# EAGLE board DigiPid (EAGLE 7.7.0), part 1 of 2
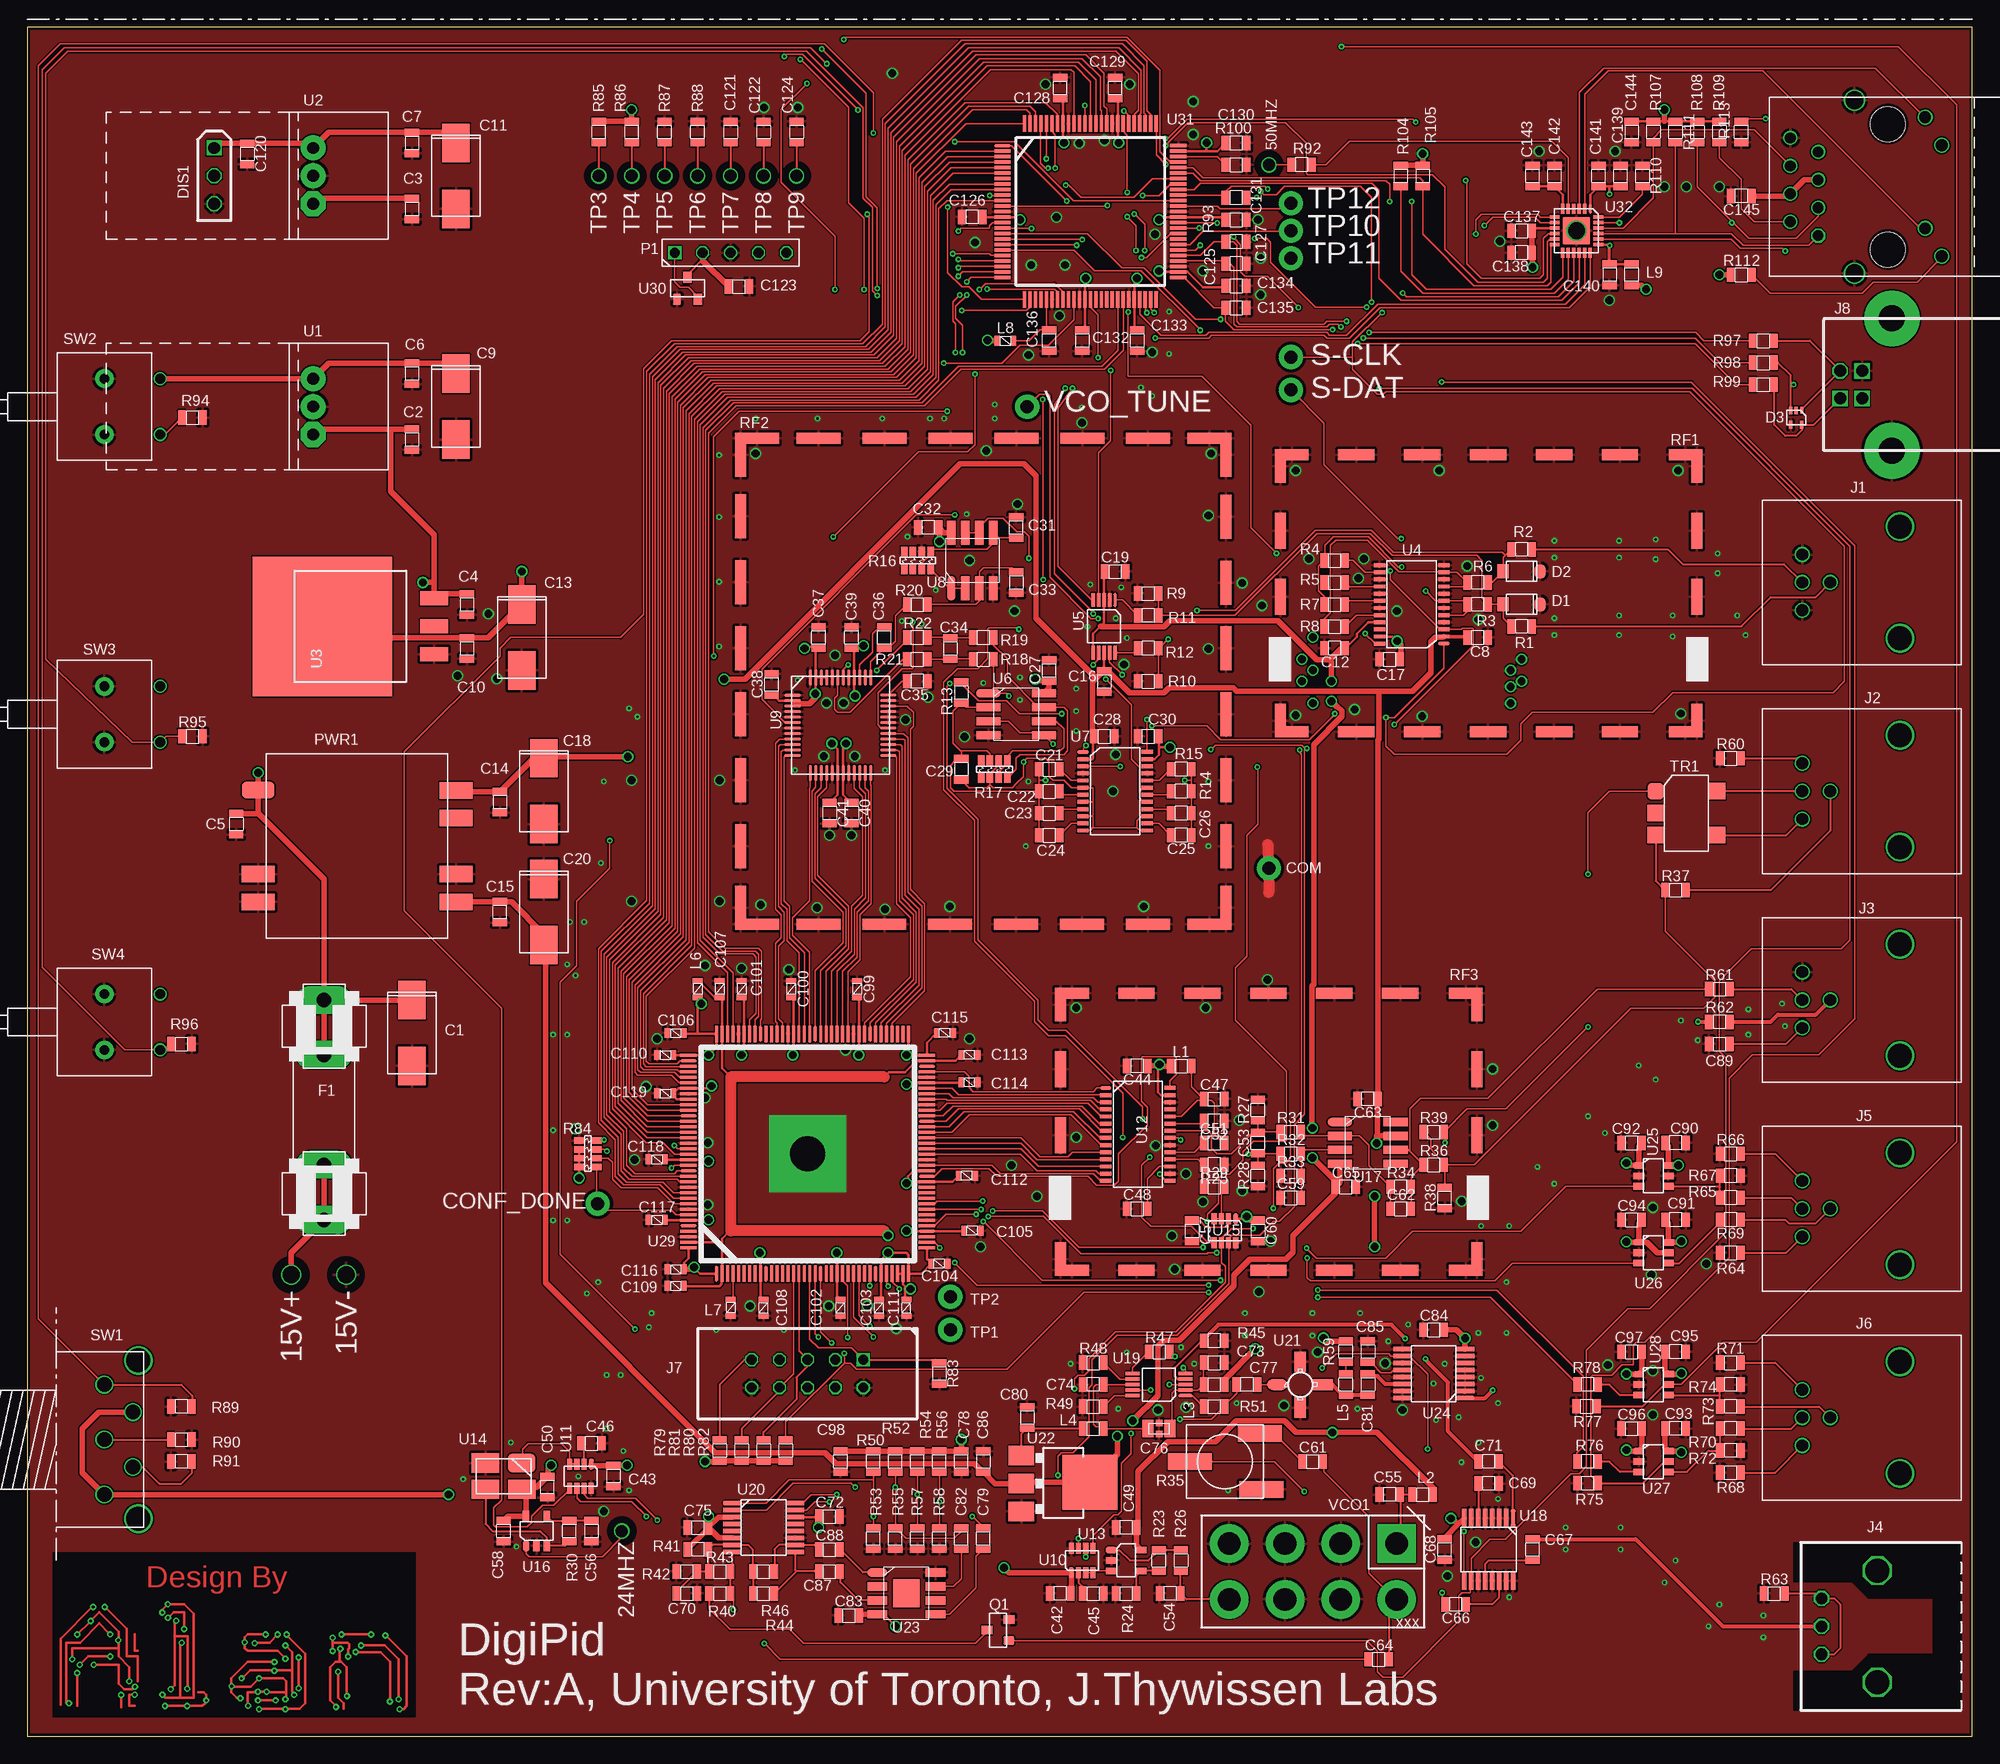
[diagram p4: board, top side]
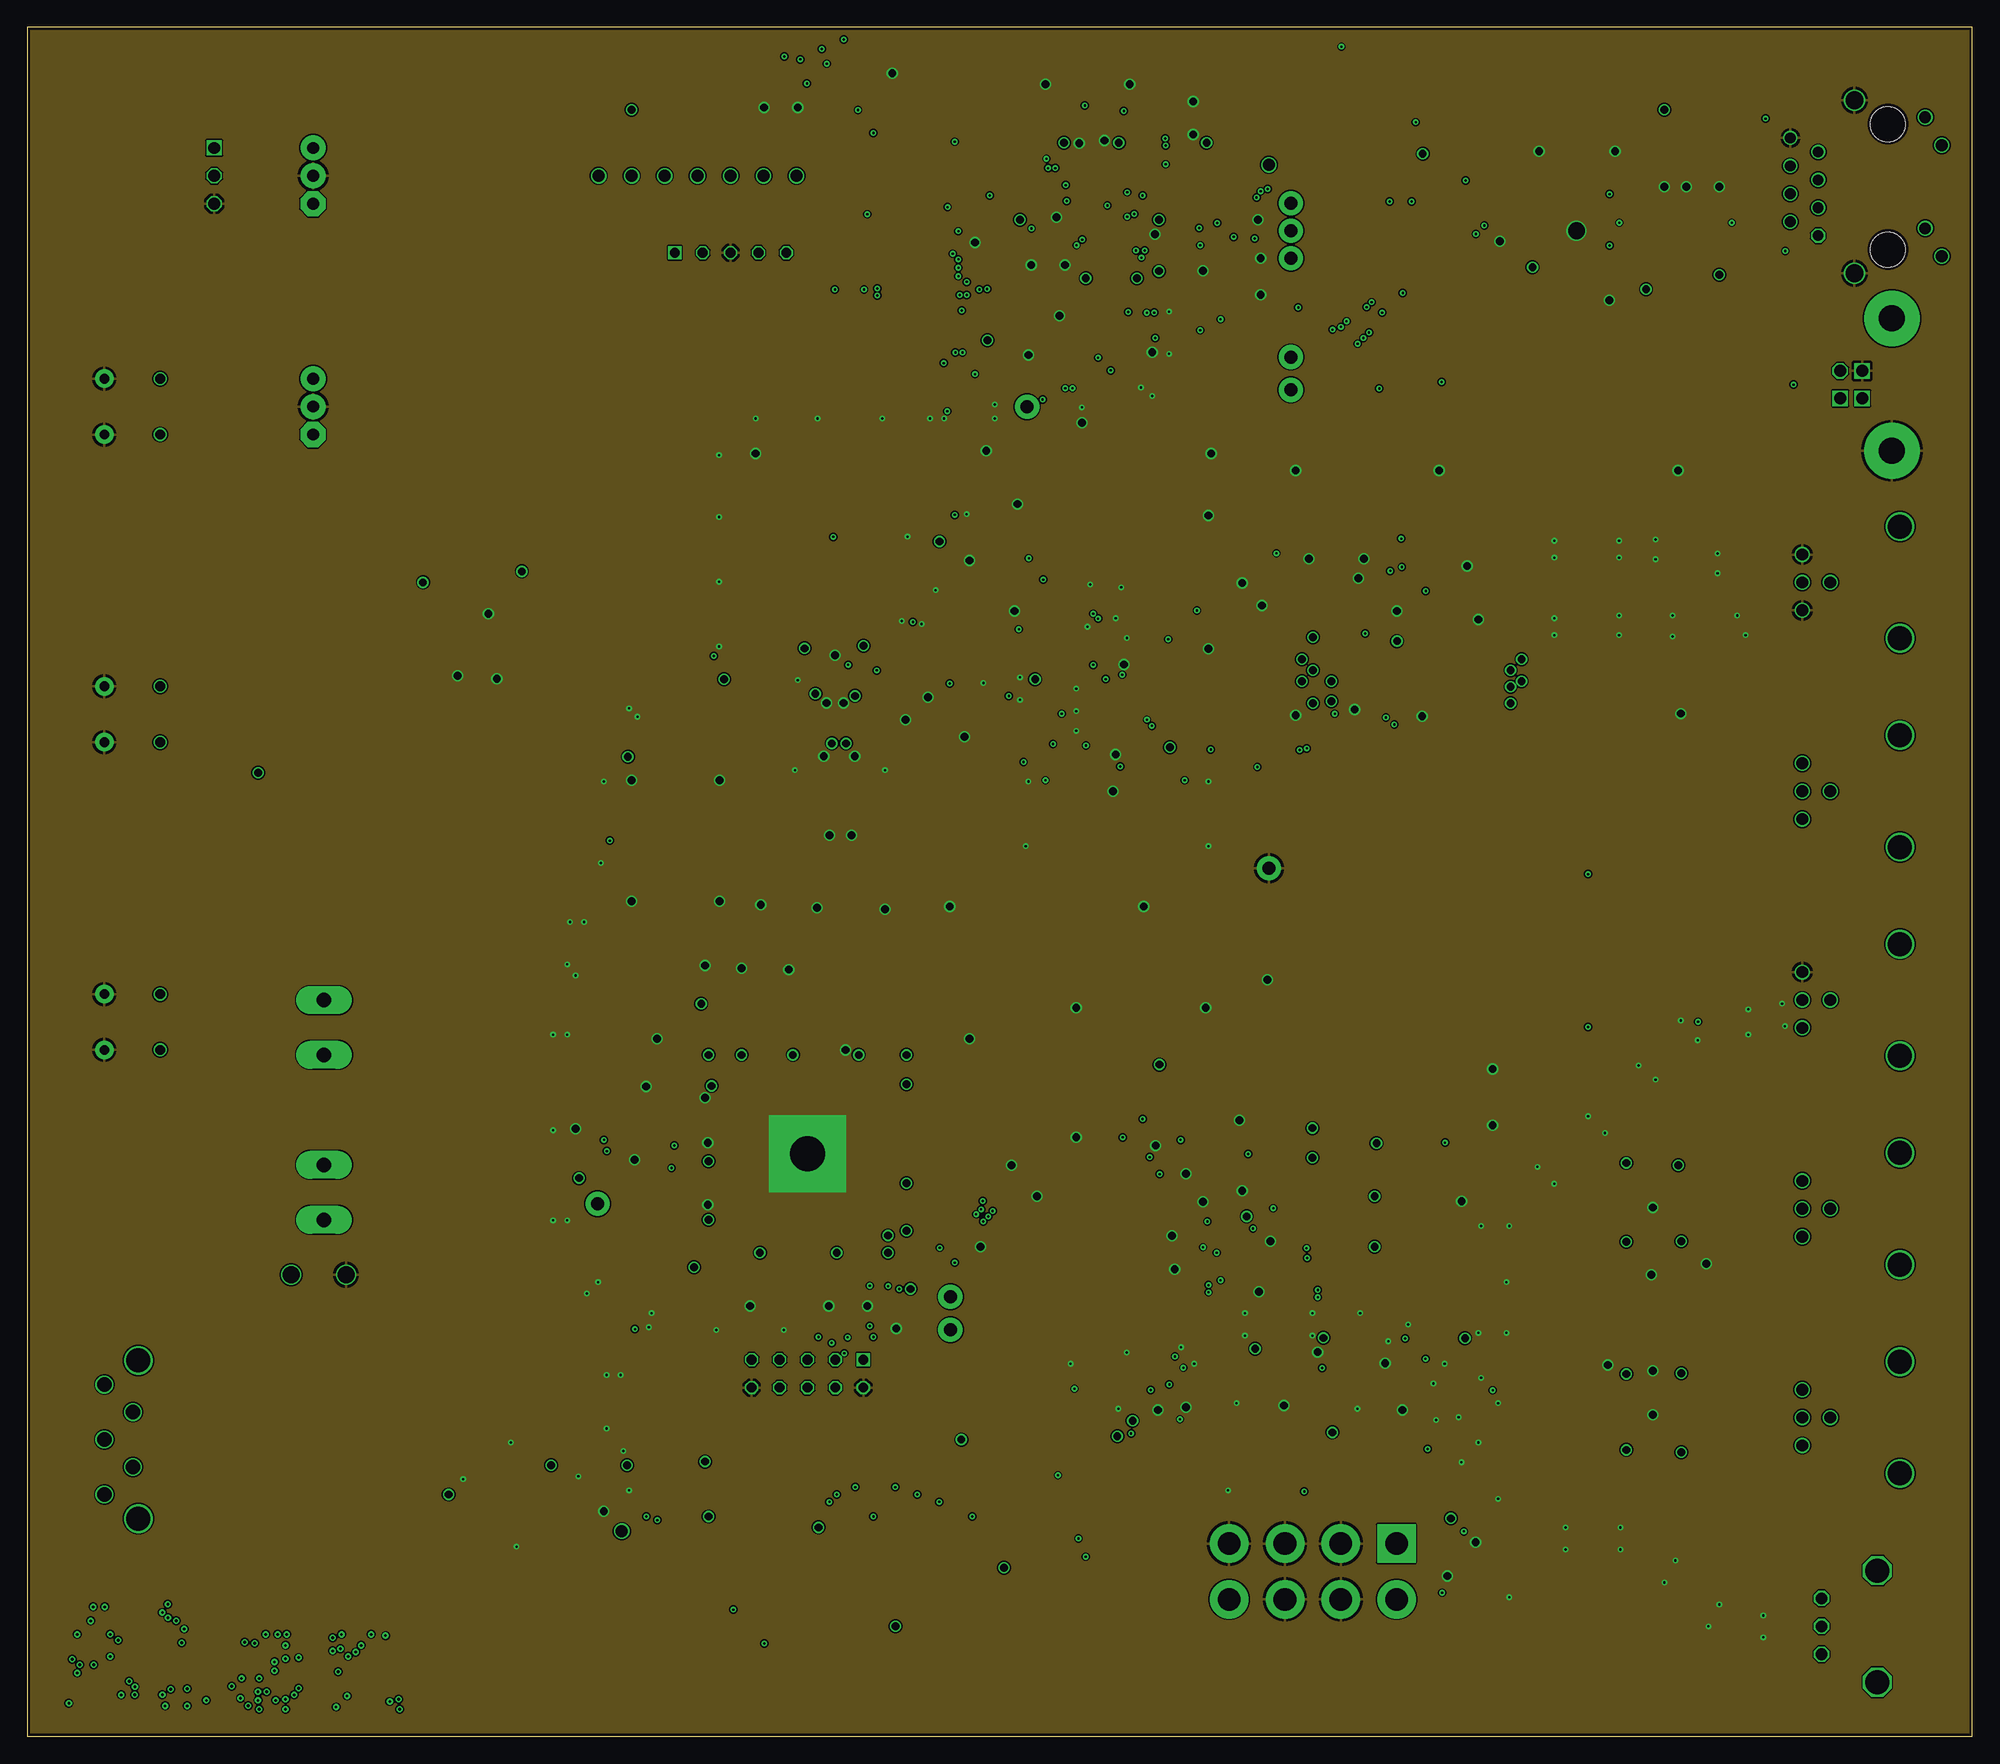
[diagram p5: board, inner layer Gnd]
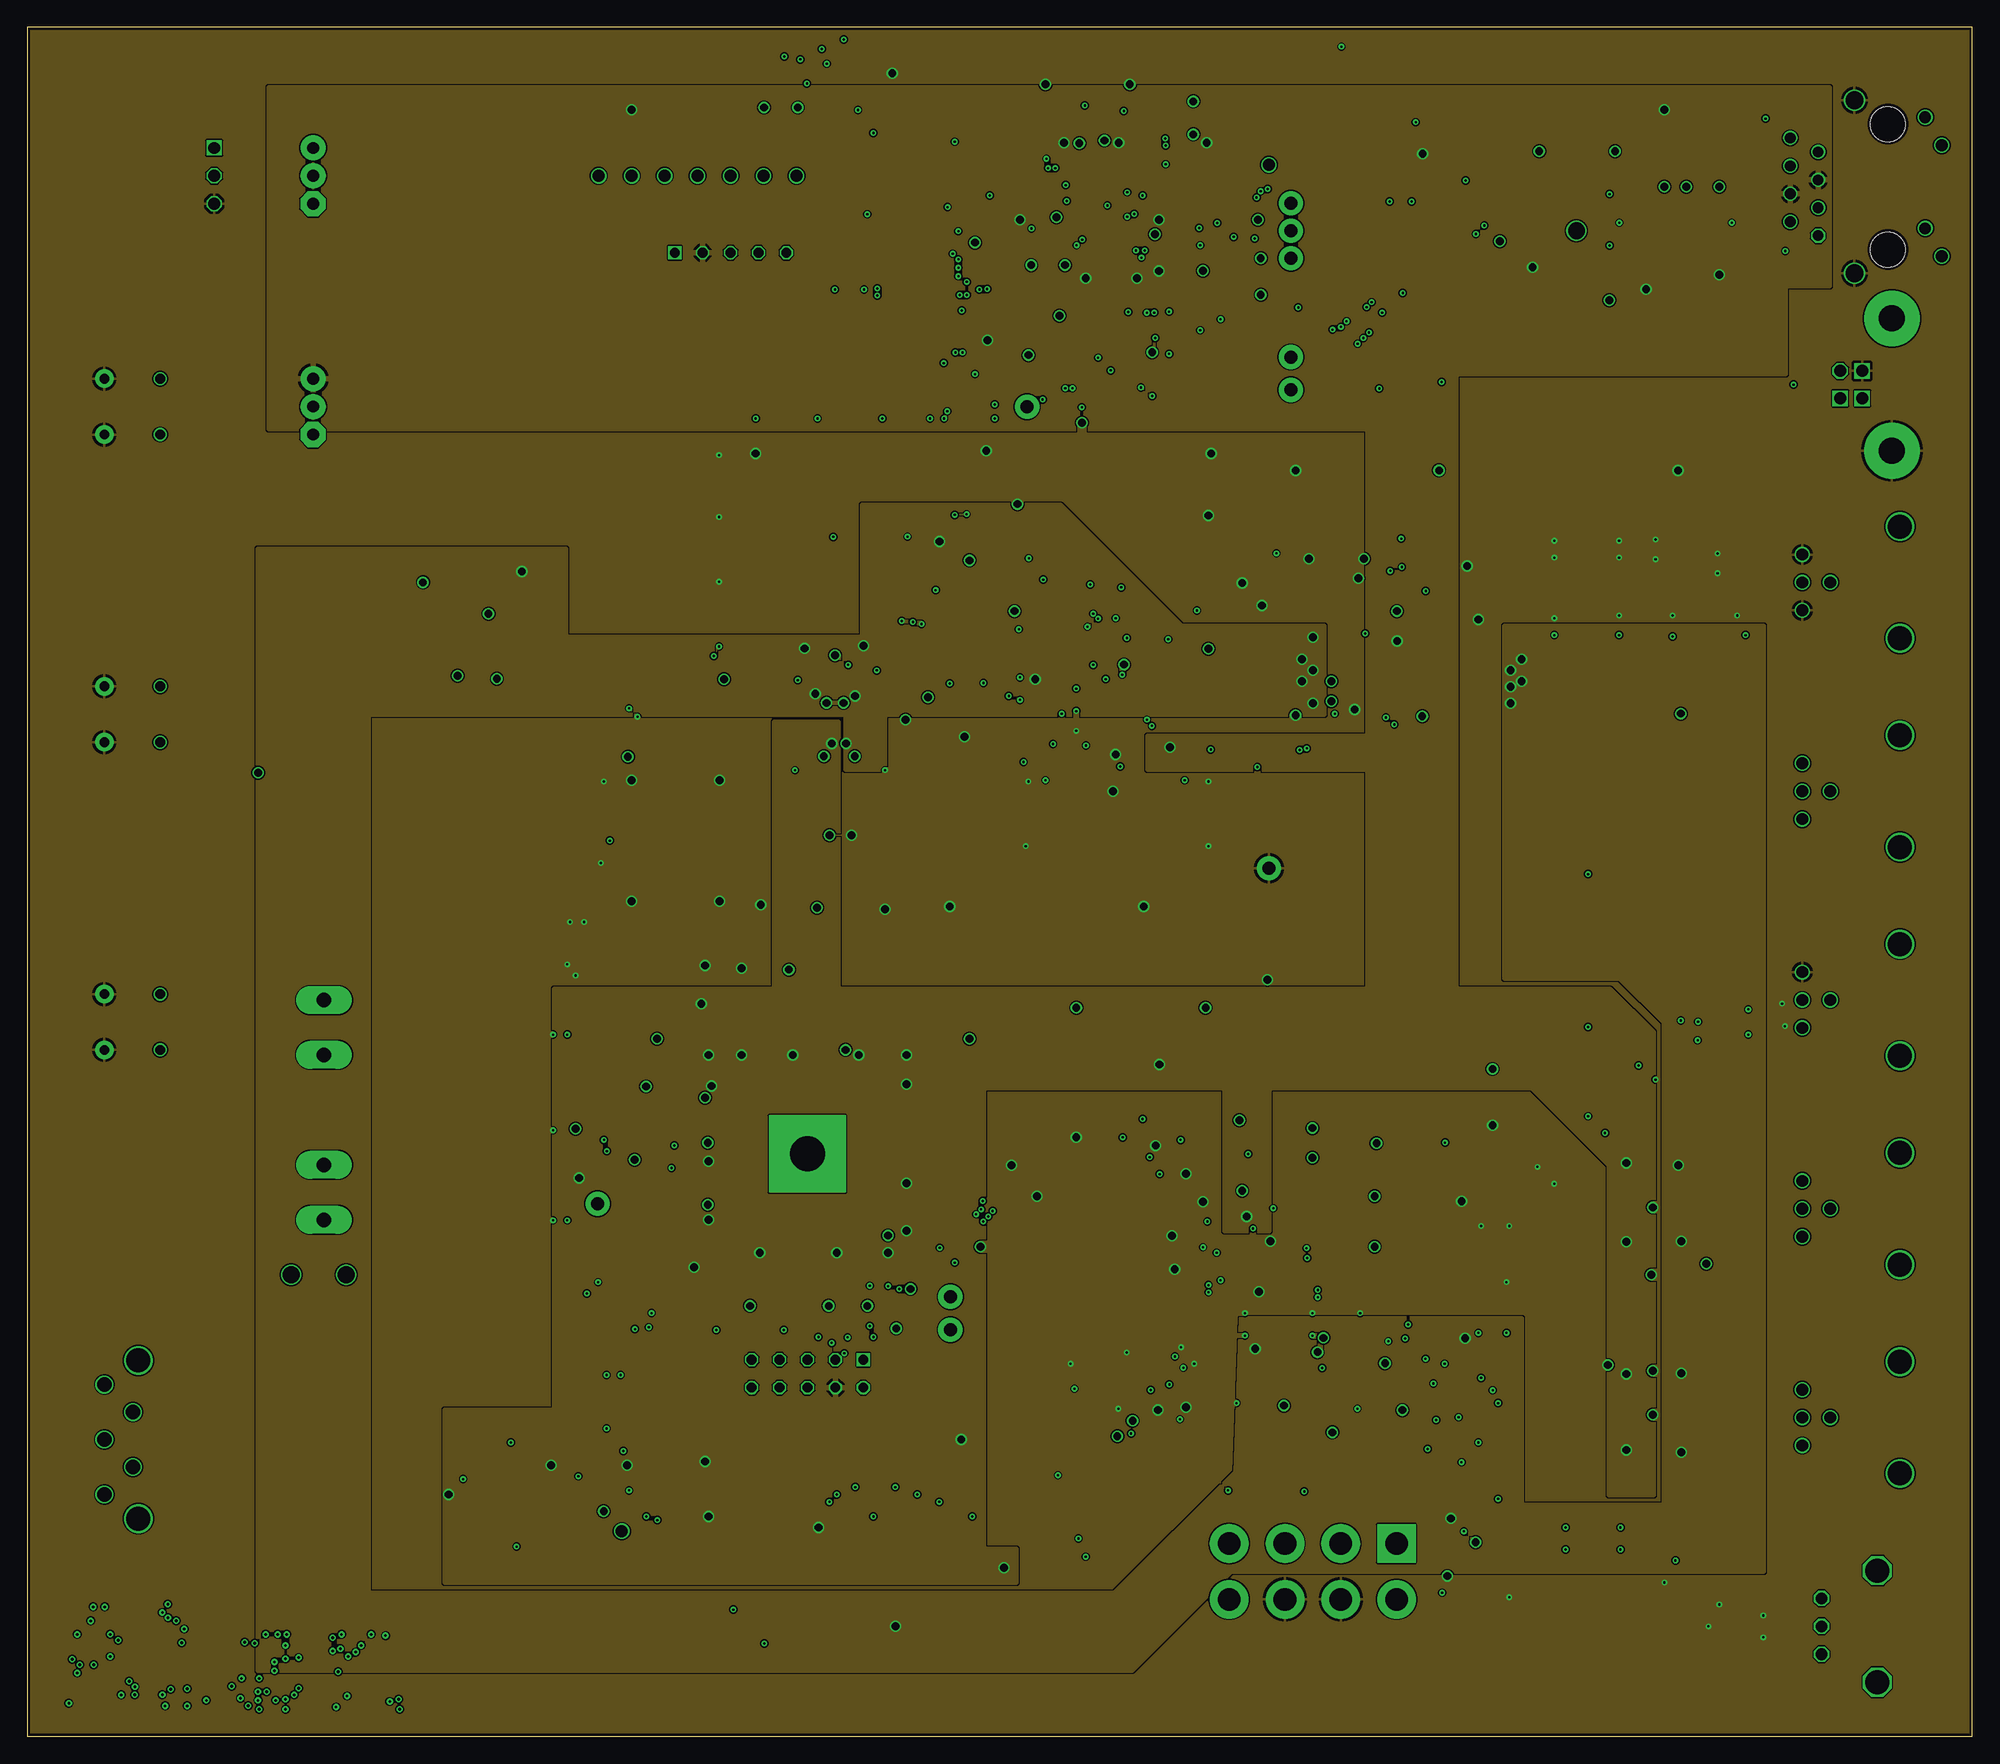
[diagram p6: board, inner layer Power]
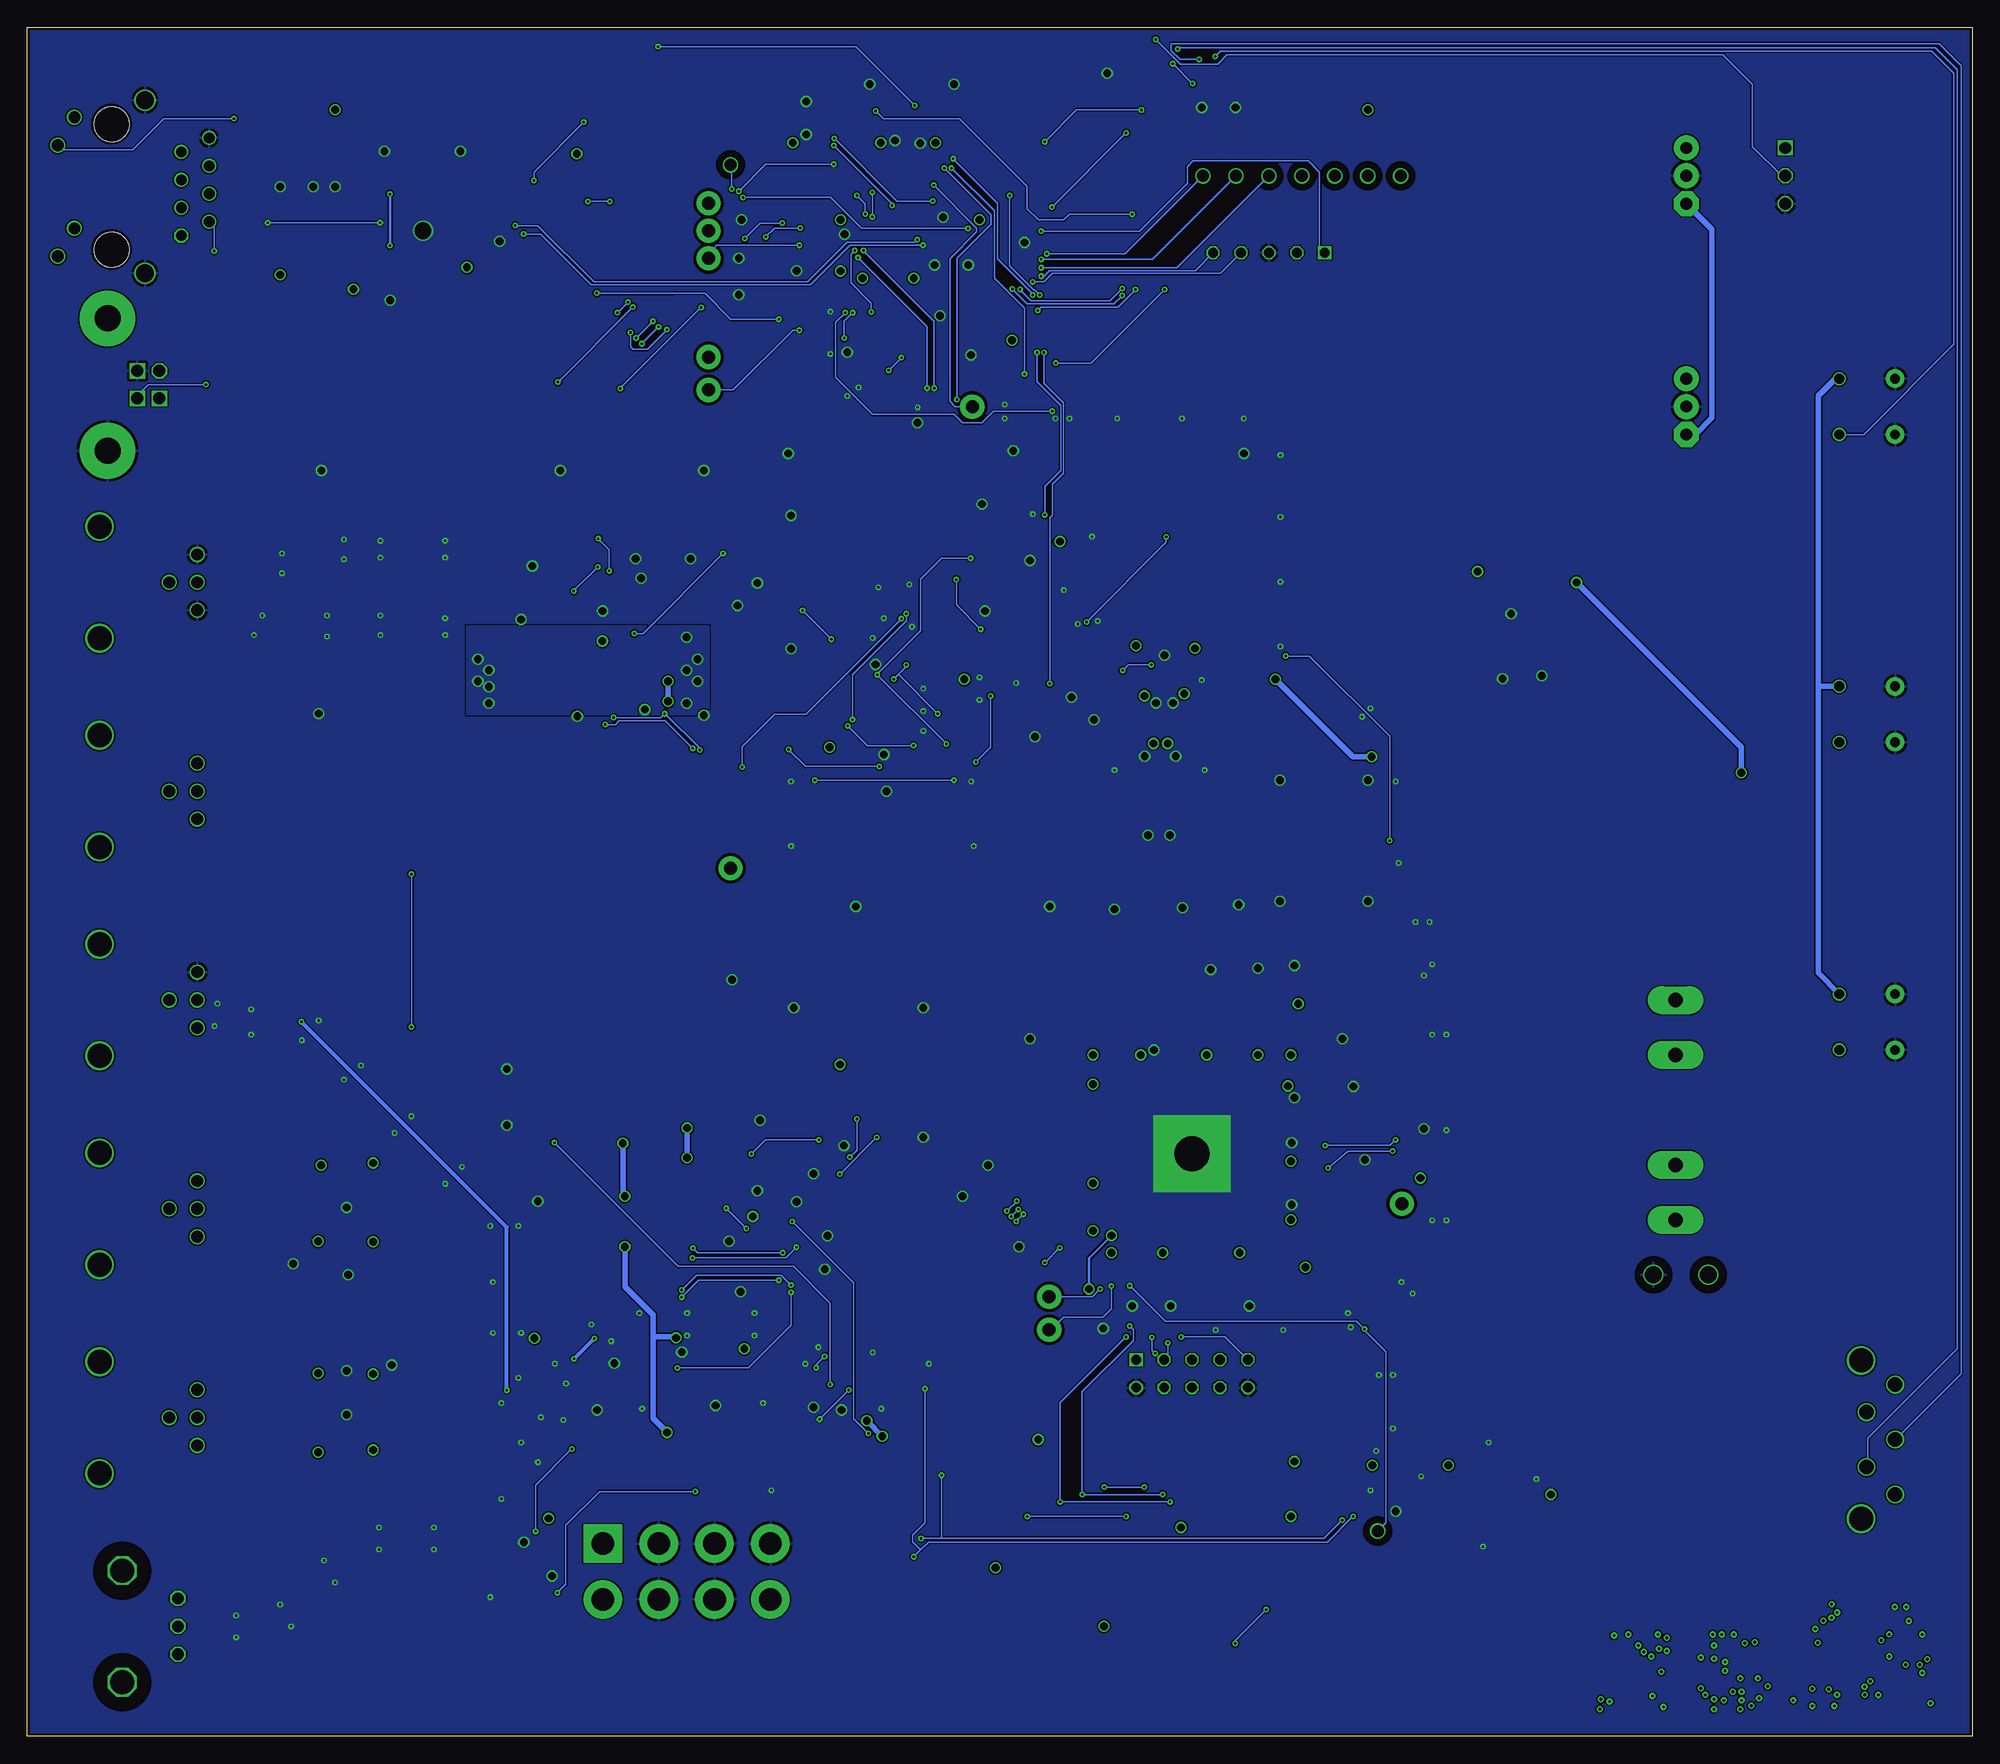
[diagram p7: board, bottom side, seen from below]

Size 177 x 155.5 mm. Coordinates in mm from the lower left corner, seen from the top.
Outline: 0,0 177,0 177,155.5 0,155.5 0,0
Copper layers (1+2+3+16): Top 0.04318125mm / dielectric 7.5mil / Gnd 0.035559375mm / dielectric 40mil / Power 0.035559375mm / dielectric 7.5mil / Bottom 0.04318125mm
Design rules "~DRC for Pentalogix, 4-layer": minimum track width 5mil, minimum drill 8mil, track to track 5mil, track to pad 5mil, pad to pad 5mil, via to via 5mil, smd to smd 0mil, copper to edge 10mil, drill to drill 5mil, minimum pad ring 6mil, minimum via ring 6mil, stop-mask expansion 4mil, vias tented up to drill 0mil, thermal gap 10mil
Net classes: 0 default: width 0.127 mm, drill 0.203 mm, clearance 0.127 mm; 1 Power: width 0.25 mm, drill 0.711 mm, clearance 0.127 mm; 2 Microstrip_50: width 0.356 mm, clearance 0.508 mm; 3 Power,0.25mm: width 0.25 mm, drill 0.711 mm, clearance 0.127 mm
tRestrict: 4 lines

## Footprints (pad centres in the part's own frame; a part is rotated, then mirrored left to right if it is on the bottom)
TP,1.5MM = drill 1.524: TP 0,0
TP-0.042B = drill 1.092: TP 0,0
7343 = smd 3.5 x 2.5: +VE -3,0; -VE 3,0
2012(0805) = smd 0.7 x 1.3: 1 -0.95,0; 2 0.95,0
1608(0603)X2Y_DUAL = smd 1 x 1.6: 1 -1,0; 2 1,0 | smd 0.6 x 0.6: COM1 0,-0.5; COM2 0,0.5
1608(0603) = smd 0.5 x 0.9: 1 -0.75,0; 2 0.75,0
TP-0.042C = drill 1.181 pad 2.2: TP 0,0
SOD123 = smd 1.016 x 1.27: A 1.676,0; C -1.676,0
SOT553 = smd 0.323 x 0.7: 1 -0.503,-0.65; 2 0,-0.65; 3 0.503,-0.65; 4 0.5,0.65; 5 -0.5,0.65
DISPLAY:3WIRE = drill 1.067 octagon: COM 0,-2.54; RXD 0,0 | drill 1.067 square: VDD 0,2.54
FUSE = drill 1.321 pad 2.54 long: 1A -10,0; 1B -5,0; 2A 10,0; 2B 5,0
CONN:BNC,DUAL(BOMAR) = drill 1.067: LWR-COM 14.45,-2.54; LWR-CTR 11.91,0; UPR-COM 14.45,2.54; UPR-CTR 14.45,0 | drill 2.184: MTG1 5.56,-5.08; MTG2 5.56,5.08
CONN:BNC-AMP-TYPE3HORIZ = drill 1.067 octagon: CONDUCTOR 0,-12.7; SHIELD1 -2.54,-12.7; SHIELD2 2.54,-12.7 | drill 2.184 octagon: P$1 -5.08,-7.62; P$2 5.08,-7.62
CONN:2X5-BLASTER = drill 0.889 square: 1 -1.27,5.08 | drill 0.889 octagon: 2 1.27,5.08; 3 -1.27,2.54; 4 1.27,2.54; 5 -1.27,0; 6 1.27,0; 7 -1.27,-2.54; 8 1.27,-2.54; 9 -1.27,-5.08; 10 1.27,-5.08
CONN,USB_AU-Y1007 = drill 1.092 octagon: 1 1.25,0 | drill 1.092 square: 2 -1.25,0; 3 -1.25,-2; 4 1.25,-2 | drill 2.362 pad 5.08: S1 -6.02,-4.71; S2 6.02,-4.71
CONN,1X5,100MIL = drill 0.889 square: 1 0,5.08 | drill 0.889 octagon: 2 0,2.54; 3 0,0; 4 0,-2.54; 5 0,-5.08
CONN,RJ45_WITH_MAGNETICS_LEDS#1 = drill 0.965 octagon: 1 4.445,0 | drill 0.965: 2 3.175,-2.54; 3 1.905,0; 4 0.635,-2.54; 5 -0.635,0; 6 -1.905,-2.54; 7 -3.175,0; 8 -4.445,-2.54 | drill 1.067: 9 6.325,11.252; 10 3.785,9.728; 11 -3.785,11.252; 12 -6.325,9.728 | drill 1.613: SHLD1 7.874,3.302; SHLD2 -7.874,3.302 | hole 3.175: 5.715,6.35; -5.715,6.35
DC-DC:CC1R5-XXXXX-R-E(TDK/LAMBDA) = smd 3 x 1.5: +VIN -9,5.1; +VOUT 9,5.08; -VIN -9,-5.08; -VOUT 9,-5.08; COM 9,-2.54; RC -9,-2.54; TRM 9,2.54
SOT23 = smd 0.75 x 1: 1 -0.95,-1; 2 0.95,-1; 3 0,1
PANASONIC_EXB-V8V(QUAD-R-PACK) = smd 0.9 x 0.59: 1A -0.8,1.2; 1B 0.8,1.2; 2A -0.8,0.4; 2B 0.8,0.4; 3A -0.8,-0.4; 3B 0.8,-0.4; 4A -0.8,-1.2; 4B 0.8,-1.2
BOURNS_3361P = smd 1.5 x 4: CCW -2.54,-3.3; CW 2.54,-3.2; W 0,3.2
RF-SHIELD,38X25MM(BMI-S-205-F) = smd 3.3 x 1: 1 -5.7,-18.95; 2 0.3,-18.95; 5 -5.7,18.95; 7 0.3,18.95 | smd 2.7 x 1: 3 6,-18.95; 8 6,18.95 | smd 3.05 x 1: 4 11.575,-18.95; 6 -11.575,18.95; 9 11.575,18.95; 25 -11.575,-18.95 | smd 1 x 3.3: 10 -12.6,-12.05; 12 -12.6,-6.05; 13 -12.6,-0.05; 15 12.6,-12.05; 17 12.6,-6.05; 18 12.6,-0.05; 20 -12.6,5.95; 21 12.6,5.95; 22 -12.6,11.95; 23 12.6,11.95 | smd 1 x 3.05: 11 -12.6,-17.925; 14 -12.6,17.925; 16 12.6,-17.925; 19 12.6,17.925
RF-SHIELD,44X44MM(BMI-S-207-F) = smd 4 x 1: 1 -15.01,-22.1; 2 -9.01,-22.1; 3 -3.01,-22.1; 4 2.99,-22.1; 5 8.99,-22.1; 6 14.99,-22.1; 13 15.01,22.1; 14 9.01,22.1; 15 3.01,22.1; 16 -2.99,22.1; 17 -8.99,22.1; 18 -14.99,22.1; 25 -20.6,-22.1; 27 20.6,-22.1; 31 -20.6,22.1; 32 20.6,22.1 | smd 1 x 4: 7 22.1,-15.01; 8 22.1,-9.01; 9 22.1,-3.01; 10 22.1,2.99; 11 22.1,8.99; 12 22.1,14.99; 19 -22.1,15.01; 20 -22.1,9.01; 21 -22.1,3.01; 22 -22.1,-2.99; 23 -22.1,-8.99; 24 -22.1,-14.99; 26 -22.1,-20.6; 28 22.1,-20.6; 29 22.1,20.6; 30 -22.1,20.6
SWITCH,QUADRATURE+PUSHSWITCH(BOURNS_PE16) = drill 1.321: A 0,-5; B 0,0; C 0,5; D -2.6,-2.5; E -2.6,2.5 | drill 2.184: MTG1 -3.1,-7.2; MTG2 -3.1,7.2
SWITCH,SPST,NKK_AB11AH = drill 0.889 pad 1.676: MTG1 0,2.54; MTG2 0,-2.54 | drill 0.889: SW1 -5.08,2.54; SW2 -5.08,-2.54
TRANSFORMER,PULSE_CX2___ = smd 1.5 x 1.5: 1 -2,-2.8; 2 0,-2.8; 3 2,-2.8; 4 2,2.8; 6 -2,2.8
TO220-SMPS = drill 1.067 pad 2.286 octagon: 1 0,2.54 | drill 1.067 pad 2.286: 2 0,0; 3 0,-2.54
TO263 = smd 1.27 x 2.54: 1 -2.54,0; 2 0,0; 3 2.54,0 | smd 12.7 x 12.7: 4 0,10.16
TSSOP-24 = smd 0.356 x 1.016: 1 -3.575,-2.925; 2 -2.925,-2.925; 3 -2.275,-2.925; 4 -1.625,-2.925; 5 -0.975,-2.925; 6 -0.325,-2.925; 7 0.325,-2.925; 8 0.975,-2.925; 9 1.625,-2.925; 10 2.275,-2.925; 11 2.925,-2.925; 12 3.575,-2.925; 13 3.575,2.925; 14 2.925,2.925; 15 2.275,2.925; 16 1.625,2.925; 17 0.975,2.925; 18 0.325,2.925; 19 -0.325,2.925; 20 -0.975,2.925; 21 -1.625,2.925; 22 -2.275,2.925; 23 -2.925,2.925; 24 -3.575,2.925
MSOP10 = smd 0.305 x 1.27: 1 -1,-2.4; 2 -0.5,-2.4; 3 0,-2.4; 4 0.5,-2.4; 5 1,-2.4; 6 1,2.4; 7 0.5,2.4; 8 0,2.4; 9 -0.5,2.4; 10 -1,2.4
SOIC-8 = smd 0.75 x 2.2: 1 -1.905,-2.532; 2 -0.635,-2.532; 3 0.635,-2.532; 4 1.905,-2.532; 5 1.905,2.532; 6 0.635,2.532; 7 -0.635,2.532; 8 -1.905,2.532
QFP48 = smd 1.5 x 0.3: 1 -4.35,2.75; 2 -4.35,2.25; 3 -4.35,1.75; 4 -4.35,1.25; 5 -4.35,0.75; 6 -4.35,0.25; 7 -4.35,-0.25; 8 -4.35,-0.75; 9 -4.35,-1.25; 10 -4.35,-1.75; 11 -4.35,-2.25; 12 -4.35,-2.75; 25 4.35,-2.75; 26 4.35,-2.25; 27 4.35,-1.75; 28 4.35,-1.25; 29 4.35,-0.75; 30 4.35,-0.25; 31 4.35,0.25; 32 4.35,0.75; 33 4.35,1.25; 34 4.35,1.75; 35 4.35,2.25; 36 4.35,2.75 | smd 0.3 x 1.5: 13 -2.75,-4.35; 14 -2.25,-4.35; 15 -1.75,-4.35; 16 -1.25,-4.35; 17 -0.75,-4.35; 18 -0.25,-4.35; 19 0.25,-4.35; 20 0.75,-4.35; 21 1.25,-4.35; 22 1.75,-4.35; 23 2.25,-4.35; 24 2.75,-4.35; 37 2.75,4.35; 38 2.25,4.35; 39 1.75,4.35; 40 1.25,4.35; 41 0.75,4.35; 42 0.25,4.35; 43 -0.25,4.35; 44 -0.75,4.35; 45 -1.25,4.35; 46 -1.75,4.35; 47 -2.25,4.35; 48 -2.75,4.35
SOT23-8 = smd 0.47 x 1: 1 -0.975,-1.1; 2 -0.325,-1.1; 3 0.325,-1.1; 4 0.975,-1.1; 5 0.975,1.1; 6 0.325,1.1; 7 -0.325,1.1; 8 -0.975,1.1
TSSOP-28 = smd 0.356 x 1.016: 1 0,-5.85; 2 0.65,-5.85; 3 1.3,-5.85; 4 1.95,-5.85; 5 2.6,-5.85; 6 3.25,-5.85; 7 3.9,-5.85; 8 4.55,-5.85; 9 5.2,-5.85; 10 5.85,-5.85; 11 6.5,-5.85; 12 7.15,-5.85; 13 7.8,-5.85; 14 8.45,-5.85; 15 8.45,0; 16 7.8,0; 17 7.15,0; 18 6.5,0; 19 5.85,0; 20 5.2,0; 21 4.55,0; 22 3.9,0; 23 3.25,0; 24 2.6,0; 25 1.95,0; 26 1.3,0; 27 0.65,0; 28 0,0
SOT23-5 = smd 0.6 x 1: 1 -0.95,-1.35; 2 0,-1.35; 3 0.95,-1.35; 4 0.95,1.35; 5 -0.95,1.35
OSCILLATOR,TAITIEN_TW_TX = smd 2.5 x 1.75: 1 -1.65,-1.2; 2 1.65,-1.2; 3 1.65,1.2; 4 -1.65,1.2
QSOP-16(RQ-16) = smd 0.406 x 1.651: 1 -2.223,-2.857; 2 -1.587,-2.857; 3 -0.953,-2.857; 4 -0.318,-2.857; 5 0.318,-2.857; 6 0.953,-2.857; 7 1.587,-2.857; 8 2.223,-2.857; 9 2.223,2.857; 10 1.587,2.857; 11 0.953,2.857; 12 0.318,2.857; 13 -0.318,2.857; 14 -0.953,2.857; 15 -1.587,2.857; 16 -2.223,2.857
MINICIRCUITS_WW107 = smd 1.016 x 1.829: 1 0,-2.083; 3 0,2.083 | smd 1.829 x 1.016: 2 2.083,0; 4 -2.083,0
SOT223 = smd 1.778 x 2.3: 1 -2.54,-2.54; 3 2.54,-2.54 | smd 1.778 x 2.286: 2 0,-2.54 | smd 5 x 5: 4 -0.1,3.7
SOIC8(E-PAD) = smd 0.75 x 1.8: 1 -1.905,-2.65; 2 -0.635,-2.65; 3 0.635,-2.65; 4 1.905,-2.65; 5 1.905,2.65; 6 0.635,2.65; 7 -0.635,2.65; 8 -1.905,2.65 | smd 2.54 x 2.413: PAD 0,0
SOT23-6 = smd 0.6 x 1: 1 -0.95,-1.35; 2 0,-1.35; 3 0.95,-1.35; 4 0.95,1.35; 5 0,1.35; 6 -0.95,1.35
EQFP144(TQFP_WITH_GROUND_PAD) = smd 1.5 x 0.27: 1 -10.89,8.29; 2 -10.89,7.79; 3 -10.89,7.29; 4 -10.89,6.79; 5 -10.89,6.29; 6 -10.89,5.79; 7 -10.89,5.29; 8 -10.89,4.79; 9 -10.89,4.29; 10 -10.89,3.79; 11 -10.89,3.29; 12 -10.89,2.79; 13 -10.89,2.29; 14 -10.89,1.79; 15 -10.89,1.29; 16 -10.89,0.79; 17 -10.89,0.29; 18 -10.89,-0.21; 19 -10.89,-0.71; 20 -10.89,-1.21; 21 -10.89,-1.71; 22 -10.89,-2.21; 23 -10.89,-2.71; 24 -10.89,-3.21; 25 -10.89,-3.71; 26 -10.89,-4.21; 27 -10.89,-4.71; 28 -10.89,-5.21; 29 -10.89,-5.71; 30 -10.89,-6.21; 31 -10.89,-6.71; 32 -10.89,-7.21; 33 -10.89,-7.71; 34 -10.89,-8.21; 35 -10.89,-8.71; 36 -10.89,-9.21; 73 10.91,-9.21; 74 10.91,-8.71; 75 10.91,-8.21; 76 10.91,-7.71; 77 10.91,-7.21; 78 10.91,-6.71; 79 10.91,-6.21; 80 10.91,-5.71; 81 10.91,-5.21; 82 10.91,-4.71; 83 10.91,-4.21; 84 10.91,-3.71; 85 10.91,-3.21; 86 10.91,-2.71; 87 10.91,-2.21; 88 10.91,-1.71; 89 10.91,-1.21; 90 10.91,-0.71; 91 10.91,-0.21; 92 10.91,0.29; 93 10.91,0.79; 94 10.91,1.29; 95 10.91,1.79; 96 10.91,2.29; 97 10.91,2.79; 98 10.91,3.29; 99 10.91,3.79; 100 10.91,4.29; 101 10.91,4.79; 102 10.91,5.29; 103 10.91,5.79; 104 10.91,6.29; 105 10.91,6.79; 106 10.91,7.29; 107 10.91,7.79; 108 10.91,8.29 | smd 0.27 x 1.5: 37 -8.54,-10.86; 38 -8.04,-10.86; 39 -7.54,-10.86; 40 -7.04,-10.86; 41 -6.54,-10.86; 42 -6.04,-10.86; 43 -5.54,-10.86; 44 -5.04,-10.86; 45 -4.54,-10.86; 46 -4.04,-10.86; 47 -3.54,-10.86; 48 -3.04,-10.86; 49 -2.54,-10.86; 50 -2.04,-10.86; 51 -1.54,-10.86; 52 -1.04,-10.86; 53 -0.54,-10.86; 54 -0.04,-10.86; 55 0.46,-10.86; 56 0.96,-10.86; 57 1.46,-10.86; 58 1.96,-10.86; 59 2.46,-10.86; 60 2.96,-10.86; 61 3.46,-10.86; 62 3.96,-10.86; 63 4.46,-10.86; 64 4.96,-10.86; 65 5.46,-10.86; 66 5.96,-10.86; 67 6.46,-10.86; 68 6.96,-10.86; 69 7.46,-10.86; 70 7.96,-10.86; 71 8.46,-10.86; 72 8.96,-10.86; 109 8.96,10.84; 110 8.46,10.84; 111 7.96,10.84; 112 7.46,10.84; 113 6.96,10.84; 114 6.46,10.84; 115 5.96,10.84; 116 5.46,10.84; 117 4.96,10.84; 118 4.46,10.84; 119 3.96,10.84; 120 3.46,10.84; 121 2.96,10.84; 122 2.46,10.84; 123 1.96,10.84; 124 1.46,10.84; 125 0.96,10.84; 126 0.46,10.84; 127 -0.04,10.84; 128 -0.54,10.84; 129 -1.04,10.84; 130 -1.54,10.84; 131 -2.04,10.84; 132 -2.54,10.84; 133 -3.04,10.84; 134 -3.54,10.84; 135 -4.04,10.84; 136 -4.54,10.84; 137 -5.04,10.84; 138 -5.54,10.84; 139 -6.04,10.84; 140 -6.54,10.84; 141 -7.04,10.84; 142 -7.54,10.84; 143 -8.04,10.84; 144 -8.54,10.84 | drill 3.175 pad 7 square: PAD 0,0
TQFP100 = smd 1.5 x 0.3: 1 -8.25,5.75; 2 -8.25,5.25; 3 -8.25,4.75; 4 -8.25,4.25; 5 -8.25,3.75; 6 -8.25,3.25; 7 -8.25,2.75; 8 -8.25,2.25; 9 -8.25,1.75; 10 -8.25,1.25; 11 -8.25,0.75; 12 -8.25,0.25; 13 -8.25,-0.25; 14 -8.25,-0.75; 15 -8.25,-1.25; 16 -8.25,-1.75; 17 -8.25,-2.25; 18 -8.25,-2.75; 19 -8.25,-3.25; 20 -8.25,-3.75; 21 -8.25,-4.25; 22 -8.25,-4.75; 23 -8.25,-5.25; 24 -8.25,-5.75; 25 -8.25,-6.25; 51 7.75,-6.25; 52 7.75,-5.75; 53 7.75,-5.25; 54 7.75,-4.75; 55 7.75,-4.25; 56 7.75,-3.75; 57 7.75,-3.25; 58 7.75,-2.75; 59 7.75,-2.25; 60 7.75,-1.75; 61 7.75,-1.25; 62 7.75,-0.75; 63 7.75,-0.25; 64 7.75,0.25; 65 7.75,0.75; 66 7.75,1.25; 67 7.75,1.75; 68 7.75,2.25; 69 7.75,2.75; 70 7.75,3.25; 71 7.75,3.75; 72 7.75,4.25; 73 7.75,4.75; 74 7.75,5.25; 75 7.75,5.75 | smd 0.3 x 1.5: 26 -6.25,-8.25; 27 -5.75,-8.25; 28 -5.25,-8.25; 29 -4.75,-8.25; 30 -4.25,-8.25; 31 -3.75,-8.25; 32 -3.25,-8.25; 33 -2.75,-8.25; 34 -2.25,-8.25; 35 -1.75,-8.25; 36 -1.25,-8.25; 37 -0.75,-8.25; 38 -0.25,-8.25; 39 0.25,-8.25; 40 0.75,-8.25; 41 1.25,-8.25; 42 1.75,-8.25; 43 2.25,-8.25; 44 2.75,-8.25; 45 3.25,-8.25; 46 3.75,-8.25; 47 4.25,-8.25; 48 4.75,-8.25; 49 5.25,-8.25; 50 5.75,-8.25; 76 5.75,7.75; 77 5.25,7.75; 78 4.75,7.75; 79 4.25,7.75; 80 3.75,7.75; 81 3.25,7.75; 82 2.75,7.75; 83 2.25,7.75; 84 1.75,7.75; 85 1.25,7.75; 86 0.75,7.75; 87 0.25,7.75; 88 -0.25,7.75; 89 -0.75,7.75; 90 -1.25,7.75; 91 -1.75,7.75; 92 -2.25,7.75; 93 -2.75,7.75; 94 -3.25,7.75; 95 -3.75,7.75; 96 -4.25,7.75; 97 -4.75,7.75; 98 -5.25,7.75; 99 -5.75,7.75; 100 -6.25,7.75
QFN24(ONE_BIG_HOLE) = smd 0.9 x 0.32: 1 -2,1.25; 2 -2,0.75; 3 -2,0.25; 4 -2,-0.25; 5 -2,-0.75; 6 -2,-1.25; 13 2,-1.25; 14 2,-0.75; 15 2,-0.25; 16 2,0.25; 17 2,0.75; 18 2,1.25 | smd 0.32 x 0.9: 7 -1.25,-2; 8 -0.75,-2; 9 -0.25,-2; 10 0.25,-2; 11 0.75,-2; 12 1.25,-2; 19 1.25,2; 20 0.75,2; 21 0.25,2; 22 -0.25,2; 23 -0.75,2; 24 -1.25,2 | smd 2.5 x 2.5: PAD 0,0 | drill 1.524: PAD-DRILL 0,0
MINICIRCUITS_A06 = drill 2.057 pad 3.5 square: 1 -7.62,-2.54 | drill 2.057 pad 3.5: 2 -7.62,2.54; 3 -2.54,-2.54; 4 -2.54,2.54; 5 2.54,-2.54; 6 2.54,2.54; 7 7.62,-2.54; 8 7.62,2.54

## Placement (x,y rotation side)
15V+  [TP,1.5MM]  24,42 270 top
15V-  [TP,1.5MM]  29,42 270 top
24MHZ  [TP-0.042B]  54.1,18.67 0 top
50MHZ  [TP-0.042B]  113,143 0 top
C1  100uF  [7343]  35,64 270 top
C2  0.1uF  [2012(0805)]  35,118 270 top
C3  0.1uF  [2012(0805)]  35,139 270 top
C4  0.1uF  [2012(0805)]  40,103 270 top
C5  0.1uF  [2012(0805)]  19,83 270 top
C6  0.1uF  [2012(0805)]  35,124 270 top
C7  0.1uF  [2012(0805)]  35,145 270 top
C8  0.1uF  [2012(0805)]  132,100 0 top
C9  100uF  [7343]  39,121 270 top
C10  0.1uF  [2012(0805)]  40,99 270 top
C11  100uF  [7343]  39,142 270 top
C12  0.1uF  [2012(0805)]  119,99 180 top
C13  100uF  [7343]  45,100 270 top
C14  0.1uF  [2012(0805)]  43,85 270 top
C15  0.1uF  [2012(0805)]  43,75 90 top
C16  0.1uF  [2012(0805)]  98,96 270 top
C17  0.1uF  [2012(0805)]  124,98 0 top
C18  100uF  [7343]  47,86 270 top
C19  0.1uF  [2012(0805)]  99,106 0 top
C20  100uF  [7343]  47,75 270 top
C21  15nF  [2012(0805)]  93,88 0 top
C22  5.1nF  [2012(0805)]  93,86 0 top
C23  1.5nF  [2012(0805)]  93,84 0 top
C24  510pF  [2012(0805)]  93,82 0 top
C25  130pF  [2012(0805)]  105,82 180 top
C26  36pF  [2012(0805)]  105,84 180 top
C27  0.1uF  [2012(0805)]  93,97 90 top
C28  0.1uF  [2012(0805)]  98,91 0 top
C29  15pF  [2012(0805)]  85,88 270 top
C30  0.1uF  [2012(0805)]  102,91 0 top
C31  0.1uF  [2012(0805)]  90,110 90 top
C32  0.1uF  [2012(0805)]  82,110 180 top
C33  0.1uF  [2012(0805)]  90,105 270 top
C34  510pF  [2012(0805)]  84,99 270 top
C35  10uF  [2012(0805)]  81,96 180 top
C36  1uF  [2012(0805)]  78,100 90 top
C37  0.1uF  [2012(0805)]  72,100 90 top
C38  0.1uF  [2012(0805)]  67.72,95.72 90 top
C39  0.1uF  [2012(0805)]  75,100 90 top
C40  0.1uF  [2012(0805)]  75,84 270 top
C41  0.1uF  [2012(0805)]  73,84 270 top
C42  0.1uF  [2012(0805)]  94,13 180 top
C43  0.1uF  [2012(0805)]  53.33,23.67 270 top
C44  0.1uF  [2012(0805)]  101,61 180 top
C45  0.1uF  [2012(0805)]  97,13 0 top
C46  0.1uF  [2012(0805)]  51.33,26.67 0 top
C47  0.1uF  [2012(0805)]  108,58 0 top
C48  0.1uF  [2012(0805)]  101,48 0 top
C49  0.1uF  [2012(0805)]  100,19 180 top
C50  0.1uF  [2012(0805)]  47.33,22.67 90 top
C51  0.1uF  [2012(0805)]  108,54 0 top
C52  0.1uF  [2012(0805)]  108,56 180 top
C53  1nF  [2012(0805)]  112,54 90 top
C54  0.1uF  [2012(0805)]  104,13 180 top
C55  0.1uF  [2012(0805)]  124,22 180 top
C56  0.1uF  [2012(0805)]  51.33,18.67 270 top
C57  0.1uF  [2012(0805)]  106,46 270 top
C58  0.1uF  [2012(0805)]  43.33,18.67 90 top
C59  47pF  [2012(0805)]  115,49 0 top
C60  0.1uF  [2012(0805)]  112,46 270 top
C61  1nF  [2012(0805)]  117,25 0 top
C62  47pF  [2012(0805)]  125,48 0 top
C63  0.1uF  [2012(0805)]  122,58 180 top
C64  1nF  [2012(0805)]  123,7 0 top
C65  0.1uF  [2012(0805)]  120,50 0 top
C66  1nF  [2012(0805)]  130,12 180 top
C67  1nF  [2012(0805)]  137,17 90 top
C68  0.1uF  [2012(0805)]  129,17 90 top
C69  1nF  [2012(0805)]  133,23 180 top
C70  0.1uF  [2012(0805)]  60,13 0 top
C71  1nF  [2012(0805)]  133,25 180 top
C72  0.1uF  [2012(0805)]  73,20 0 top
C73  2.2uF  [2012(0805)]  108,34 0 top
C74  2.2uF  [2012(0805)]  97,32 180 top
C75  0.1uF  [2012(0805)]  61,19 0 top
C76  0.1uF  [1608(0603)X2Y_DUAL]  103,28 0 top
C77  1nF  [2012(0805)]  111,32 180 top
C78  0.1uF  [2012(0805)]  85,25 90 top
C79  1nF  [2012(0805)]  87,18 90 top
C80  0.1uF  [2012(0805)]  91,29 270 top
C81  1nF  [2012(0805)]  122,32 270 top
C82  1nF  [2012(0805)]  85,18 90 top
C83  0.1uF  [2012(0805)]  74.74,11 0 top
C84  0.1uF  [2012(0805)]  128,37 0 top
C85  1nF  [2012(0805)]  122,35 270 top
C86  0.1uF  [2012(0805)]  87,25 270 top
C87  1nF  [2012(0805)]  73,15 0 top
C88  1nF  [2012(0805)]  73,17 0 top
C89  1nF  [2012(0805)]  154,65 180 top
C90  0.1uF  [2012(0805)]  150,54 180 top
C91  0.1uF  [2012(0805)]  150,47 180 top
C92  0.1uF  [2012(0805)]  146,54 0 top
C93  0.1uF  [2012(0805)]  150,28 180 top
C94  0.1uF  [2012(0805)]  146,47 0 top
C95  0.1uF  [2012(0805)]  150,35 180 top
C96  0.1uF  [2012(0805)]  146,28 0 top
C97  0.1uF  [2012(0805)]  146,35 0 top
C98  0.1uF  [2012(0805)]  74,25 90 top
C99  0.1uF  [1608(0603)]  75.5,68 270 top
C100  0.1uF  [1608(0603)]  69.5,68 270 top
C101  0.1uF  [1608(0603)]  65,68 270 top
C102  0.1uF  [1608(0603)]  74,39 90 top
C103  0.1uF  [1608(0603)]  77.5,39 90 top
C104  0.1uF  [1608(0603)]  83,43 180 top
C105  0.1uF  [1608(0603)]  86,46 180 top
C106  0.1uF  [1608(0603)]  59,64 0 top
C107  0.1uF  [1608(0603)]  63,68 270 top
C108  0.1uF  [1608(0603)]  67,39 90 top
C109  0.1uF  [1608(0603)]  59,41 0 top
C110  0.1uF  [1608(0603)]  58.05,62 0 top
C111  0.1uF  [1608(0603)]  80,39 90 top
C112  0.1uF  [1608(0603)]  85.5,51 180 top
C113  0.1uF  [1608(0603)]  85.74,62 180 top
C114  0.1uF  [1608(0603)]  85.74,59.5 180 top
C115  0.1uF  [1608(0603)]  83.5,64 180 top
C116  0.1uF  [1608(0603)]  59,42.5 0 top
C117  0.1uF  [1608(0603)]  57.28,47 0 top
C118  0.1uF  [1608(0603)]  57.28,52.51 0 top
C119  0.1uF  [1608(0603)]  58.05,58.5 0 top
C120  0.1uF  [2012(0805)]  20,144 270 top
C121  0.1uF  [2012(0805)]  64,146 270 top
C122  0.1uF  [2012(0805)]  67,146 270 top
C123  0.1uF  [2012(0805)]  64.77,131.93 0 top
C124  0.1uF  [2012(0805)]  70,146 270 top
C125  out  [2012(0805)]  110,134 180 top
C126  0.1uF  [2012(0805)]  86,138.26 180 top
C127  out  [2012(0805)]  110,136 180 top
C128  0.1uF  [2012(0805)]  94,150 90 top
C129  0.1uF  [2012(0805)]  99,150 90 top
C130  0.1uF  [2012(0805)]  110,145 0 top
C131  0.1uF  [2012(0805)]  110,138 0 top
C132  0.1uF  [2012(0805)]  96,127 270 top
C133  0.1uF  [2012(0805)]  101,127 270 top
C134  0.1uF  [2012(0805)]  110,132 0 top
C135  0.1uF  [2012(0805)]  110,130 0 top
C136  0.1uF  [2012(0805)]  93,127 90 top
C137  1nF  [2012(0805)]  136,137 0 top
C138  0.1uF  [2012(0805)]  136,135 180 top
C139  0.1uF  [2012(0805)]  145,142 90 top
C140  1nF  [2012(0805)]  144,133 270 top
C141  1nF  [2012(0805)]  143,142 90 top
C142  1nF  [2012(0805)]  139,142 90 top
C143  1uF  [2012(0805)]  137,142 90 top
C144  0.1uF  [2012(0805)]  146,146 270 top
C145  0.1uF  [2012(0805)]  156,140.16 180 top
COM  [TP-0.042C]  113,79 0 top
CONF_DONE  [TP-0.042C]  51.91,48.45 180 top
D1  ATV02W120B-HF  [SOD123]  136,103 180 top
D2  ATV02W120B-HF  [SOD123]  136,106 180 top
D3  TPD2E001DRLR  [SOT553]  161,120 180 top
DIS1  NHD-0220D3Z-FL-GBW-V3  [DISPLAY:3WIRE]  17,142 0 top
F1  ???A  [FUSE]  27,57 90 top
J1  031-6575  [CONN:BNC,DUAL(BOMAR)]  176,105 180 top
J2  031-6575  [CONN:BNC,DUAL(BOMAR)]  176,86 180 top
J3  031-6575  [CONN:BNC,DUAL(BOMAR)]  176,67 180 top
J4  5227677-1  [CONN:BNC-AMP-TYPE3HORIZ]  176,10 270 top
J5  031-6575  [CONN:BNC,DUAL(BOMAR)]  176,48 180 top
J6  031-6575  [CONN:BNC,DUAL(BOMAR)]  176,29 180 top
J7  XG4C-1031  [CONN:2X5-BLASTER]  71,33 270 top
J8  AU-Y1007  [CONN,USB_AU-Y1007]  165,123 90 top
L1  BLM21PG221SN1D  [2012(0805)]  105,61 0 top
L2  BLM21PG221SN1D  [2012(0805)]  127,22 0 top
L3  BLM21PG221SN1D  [2012(0805)]  108,32 0 top
L4  BLM21PG221SN1D  [2012(0805)]  97,28 0 top
L5  BLM21PG221SN1D  [2012(0805)]  120,32 90 top
L6  BLM18BB221  [1608(0603)]  61,68 270 top
L7  BLM18BB221  [1608(0603)]  64,39 270 top
L8  BLM18HK102SN1D  [1608(0603)]  89,127 0 top
L9  BLM21PG221SN1D  [2012(0805)]  146,133 270 top
P1  61300511121  [CONN,1X5,100MIL]  64,135 90 top
P2  J00-0045NL  [CONN,RJ45_WITH_MAGNETICS_LEDS#1]  163,141 270 top
PWR1  CC1R5-1212DR-E  [DC-DC:CC1R5-XXXXX-R-E(TDK/LAMBDA)]  30,81 0 top
Q1  2N7002-TP  [SOT23]  88.33,9.67 90 top
R1  4.99  [2012(0805)]  136,101 180 top
R2  4.99  [2012(0805)]  136,108 180 top
R3  40.2  [2012(0805)]  132,103 180 top
R4  1K  [2012(0805)]  119,107 0 top
R5  1K  [2012(0805)]  119,105 0 top
R6  40.2  [2012(0805)]  132,105 180 top
R7  10K  [2012(0805)]  119,103 0 top
R8  10K  [2012(0805)]  119,101 0 top
R9  1M  [2012(0805)]  102,104 0 top
R10  1M  [2012(0805)]  102,96 0 top
R11  1K  [2012(0805)]  102,102 180 top
R12  1K  [2012(0805)]  102,99 180 top
R13  24.9K  [2012(0805)]  85,95 270 top
R14  6.19K  [2012(0805)]  105,86 180 top
R15  24.9K  [2012(0805)]  105,88 180 top
R16  10K  [PANASONIC_EXB-V8V(QUAD-R-PACK)]  81,107 270 top
R17  10K  [PANASONIC_EXB-V8V(QUAD-R-PACK)]  88,88 270 top
R18  10  [2012(0805)]  87,98 0 top
R19  10  [2012(0805)]  87,100 0 top
R20  10K  [2012(0805)]  81,103 0 top
R21  49.9  [2012(0805)]  81,98 0 top
R22  49.9  [2012(0805)]  81,100 0 top
R23  38.3K  [2012(0805)]  103,16 90 top
R24  10K  [2012(0805)]  100,13 0 top
R25  3.32K  [2012(0805)]  108,52 180 top
R26  10K  [2012(0805)]  105,16 270 top
R27  49.9  [2012(0805)]  112,57 90 top
R28  49.9  [2012(0805)]  112,51 90 top
R29  4.42K  [2012(0805)]  108,50 0 top
R30  10K  [2012(0805)]  49.33,18.67 90 top
R31  100  [2012(0805)]  115,55 0 top
R32  100  [2012(0805)]  115,53 0 top
R33  1.5K  [2012(0805)]  115,51 0 top
R34  1.5K  [2012(0805)]  125,50 0 top
R35  100  [BOURNS_3361P]  109,25 90 top
R36  604  [2012(0805)]  128,52 0 top
R37  1K  [2012(0805)]  150,77 0 top
R38  100  [2012(0805)]  129,49 90 top
R39  100  [2012(0805)]  128,55 0 top
R40  1K  [2012(0805)]  63,13 0 top
R41  1K  [2012(0805)]  61,17 180 top
R42  1K  [2012(0805)]  60,15 0 top
R43  1K  [2012(0805)]  63,15 0 top
R44  1K  [2012(0805)]  67,13 0 top
R45  100  [2012(0805)]  108,36 180 top
R46  1K  [2012(0805)]  67,15 0 top
R47  453  [2012(0805)]  103,35 0 top
R48  100  [2012(0805)]  97,34 0 top
R49  20  [2012(0805)]  97,30 0 top
R50  127  [2012(0805)]  77,25 90 top
R51  453  [2012(0805)]  108,30 0 top
R52  127  [2012(0805)]  79,25 90 top
R53  82.5  [2012(0805)]  77,18 90 top
R54  127  [2012(0805)]  81,25 90 top
R55  82.5  [2012(0805)]  79,18 90 top
R56  127  [2012(0805)]  83,25 90 top
R57  82.5  [2012(0805)]  81,18 90 top
R58  82.5  [2012(0805)]  83,18 90 top
R59  100  [2012(0805)]  120,35 90 top
R60  4.99  [2012(0805)]  155,89 0 top
R61  49.9  [2012(0805)]  154,68 0 top
R62  4.99  [2012(0805)]  154,63 0 top
R63  4.99  [2012(0805)]  159,13 0 top
R64  4.99  [2012(0805)]  155,44 0 top
R65  49.9  [2012(0805)]  155,49 180 top
R66  4.99  [2012(0805)]  155,53 0 top
R67  10K  [2012(0805)]  155,51 180 top
R68  4.99  [2012(0805)]  155,24 0 top
R69  49.9  [2012(0805)]  155,47 180 top
R70  49.9  [2012(0805)]  155,28 180 top
R71  4.99  [2012(0805)]  155,34 0 top
R72  10K  [2012(0805)]  155,26 180 top
R73  49.9  [2012(0805)]  155,30 180 top
R74  10K  [2012(0805)]  155,32 180 top
R75  10K  [2012(0805)]  142.01,23.04 0 top
R76  1K  [2012(0805)]  142,25 180 top
R77  10K  [2012(0805)]  141.93,30.04 0 top
R78  1K  [2012(0805)]  142,32 180 top
R79  10K  [2012(0805)]  63,26 270 top
R80  10K  [2012(0805)]  67,26 270 top
R81  10K  [2012(0805)]  65,26 270 top
R82  10K  [2012(0805)]  69,26 270 top
R83  1K  [2012(0805)]  83,33 270 top
R84  10K  [PANASONIC_EXB-V8V(QUAD-R-PACK)]  51,53 0 top
R85  49.9  [2012(0805)]  52,146 90 top
R86  49.9  [2012(0805)]  55,146 90 top
R87  49.9  [2012(0805)]  58,146 90 top
R88  49.9  [2012(0805)]  61,146 90 top
R89  10K  [2012(0805)]  14,30 180 top
R90  10K  [2012(0805)]  14,27 0 top
R91  10K  [2012(0805)]  14,25 180 top
R92  30.1  [2012(0805)]  116,143 180 top
R93  30.1  [2012(0805)]  110,140 180 top
R94  10K  [2012(0805)]  15,120 0 top
R95  10K  [2012(0805)]  15,91 0 top
R96  10K  [2012(0805)]  14,63 0 top
R97  100  [2012(0805)]  158,127 0 top
R98  30.1  [2012(0805)]  158,125 0 top
R99  30.1  [2012(0805)]  158,123 0 top
R100  1K  [2012(0805)]  110,143 0 top
R104  4.7K  [2012(0805)]  125,142 270 top
R105  1.5K  [2012(0805)]  127,142 270 top
R107  49.9  [2012(0805)]  148,146 270 top
R108  49.9  [2012(0805)]  152,146 270 top
R109  49.9  [2012(0805)]  154,146 270 top
R110  12.1K  [2012(0805)]  147,142 270 top
R111  49.9  [2012(0805)]  150,146 270 top
R112  249  [2012(0805)]  156,133 0 top
R113  249  [2012(0805)]  156,146 90 top
RF1  BMI-S-205-F  [RF-SHIELD,38X25MM(BMI-S-205-F)]  133,104 270 top
RF2  BMI-S-207-F  [RF-SHIELD,44X44MM(BMI-S-207-F)]  87,96 0 top
RF3  BMI-S-205-F  [RF-SHIELD,38X25MM(BMI-S-205-F)]  113,55 270 top
S-CLK  [TP-0.042C]  115,125.51 0 top
S-DAT  [TP-0.042C]  115,122.51 0 top
SW1  PEC16-2220F-S0024  [SWITCH,QUADRATURE+PUSHSWITCH(BOURNS_PE16)]  7,27 180 top
SW2  AB11AH-HA  [SWITCH,SPST,NKK_AB11AH]  7,121 180 top
SW3  AB11AH-HA  [SWITCH,SPST,NKK_AB11AH]  7,93 180 top
SW4  AB11AH-HA  [SWITCH,SPST,NKK_AB11AH]  7,65 180 top
TP1  [TP-0.042C]  84,37 0 top
TP2  [TP-0.042C]  84,40 0 top
TP3  [TP-0.042B]  52,142 270 top
TP4  [TP-0.042B]  55,142 270 top
TP5  [TP-0.042B]  58,142 270 top
TP6  [TP-0.042B]  61,142 270 top
TP7  [TP-0.042B]  64,142 270 top
TP8  [TP-0.042B]  67,142 270 top
TP9  [TP-0.042B]  70,142 270 top
TP10  [TP-0.042C]  115,137 0 top
TP11  [TP-0.042C]  115,134.49 0 top
TP12  [TP-0.042C]  115,139.51 0 top
TR1  CX2147NL  [TRANSFORMER,PULSE_CX2___]  151,84 270 top
U1  P78A03-1000  [TO220-SMPS]  26,121 180 top
U2  P78A03-1000  [TO220-SMPS]  26,142 180 top
U3  LM1086ISX-5  [TO263]  37,101 90 top
U4  ADG1414BRU  [TSSOP-24]  126,103 90 top
U5  AD8253ARM  [MSOP10]  98,101 180 top
U6  AD8656AR  [SOIC-8]  90,93 270 top
U7  ADG1414BRU  [TSSOP-24]  99,86 270 top
U8  AD8656AR  [SOIC-8]  86,107 0 top
U9  LTC2389CLX-16  [QFP48]  74,92 0 top
U10  AD5660BRJZ-2500  [SOT23-8]  96,16 0 top
U11  AD5620ARJZ-2500  [SOT23-8]  50.33,23.67 180 top
U12  AD9764ARUZ  [TSSOP-28]  104,59 270 top
U13  AD8638ARJ  [SOT23-5]  100,16 270 top
U14  TXEABLSANF-24.0  [OSCILLATOR,TAITIEN_TW_TX]  43.33,23.67 180 top
U15  AD5620ARJZ-2500  [SOT23-8]  109,46 180 top
U16  ADCMP600BRJZ  [SOT23-5]  46.33,18.67 0 top
U17  AD8627ARZ  [SOIC-8]  122,54 270 top
U18  HMC245AQS16E  [QSOP-16(RQ-16)]  133,17 180 top
U19  VCA821IDGS  [MSOP10]  103,32 90 top
U20  ADCMP551BRQ  [QSOP-16(RQ-16)]  67,19 270 top
U21  ERA-6SM  [MINICIRCUITS_WW107]  115.85,32 270 top
U22  LT1175CST-5  [SOT223]  93,23 270 top
U23  HMC361S8G  [SOIC8(E-PAD)]  80,13 270 top
U24  HMC245AQS16E  [QSOP-16(RQ-16)]  128,33 90 top
U25  SN74LVC1T45DBV  [SOT23-6]  148,51 270 top
U26  SN74LVC1T45DBV  [SOT23-6]  148,44 270 top
U27  SN74LVC1T45DBV  [SOT23-6]  148,25 270 top
U28  SN74LVC1T45DBV  [SOT23-6]  148,32 270 top
U29  10M08SAE144I7G  [EQFP144(TQFP_WITH_GROUND_PAD)]  71,53 90 top
U30  MIC803-40D4VM3  [SOT23]  60.07,131.76 0 top
U31  PIC32MZ1024EFE100-I/PF  [TQFP100]  97,139 0 top
U32  LAN8720A  [QFN24(ONE_BIG_HOLE)]  141,137 270 top
U$191  [CASE:HAMMOND_1402DV]  0,0 0 top
VCO1  Minicircuits A06  [MINICIRCUITS_A06]  117,15 180 top
VCO_TUNE  [TP-0.042C]  91,121 0 top

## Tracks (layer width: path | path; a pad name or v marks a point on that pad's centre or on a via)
24MHZ  (via drill 0.2)
  Top 0.127: U29.29 76.71,41.04 v76.67,41 | U16.1 45.38,16.62 45.67,16.33 52.33,16.33 54.1,18.1 24MHZ.TP | U31.49 102.25,129.85 v102.55,129.55 | v55.3,37.05 48.5,43.85 48.5,68.6 50,70.1 50,76 53,79 v53,81.5 | v83.71,120.58 64.77,120.58 62.46,118.27 62.46,98.8 v62.47,98.3
  Bottom 0.127: v76.67,41 73.44,37.77 56.02,37.77 v55.3,37.05 55.33,37 53.33,35 53.33,19.43 24MHZ.TP | v62.47,98.3 60.3,98.3 53,91 v53,81.5 | v102.55,129.55 103.42,128.68 103.42,123.65 100.1,120.32 92.67,120.32 91.9,119.55 90.11,119.55 89.09,120.58 v83.71,120.58
50MHZ_MAC  (via drill 0.2)
  Top 0.127: U31.16 91.36,137.25 v91.39,137.22 | R93.1 111.84,140 v111.87,140.03
  Bottom 0.127: v91.39,137.22 101.1,137.22 103.91,140.03 v111.87,140.03
!ADC-CNVST
  Top 0.127: U9.34 80.07,93.75 80.64,93.18 80.64,91.9 80.38,91.65 80.38,77.06 81.66,75.78 81.66,67.84 78.71,64.89 U29.76
!BW_CTRL  (via drill 0.2)
  Top 0.127: v101.9,92.51 101.9,89.6 U7.24 | v97,102.15 97,102.3 93.5,105.8 93.5,121.19 v94.47,122.67 | v100.9,135.2 100.9,137.48 v100.1,138.28 | v100.1,140.5 100.1,145.7 99.75,146.05 U31.82
  Bottom 0.127: v101.9,92.51 101.9,96.6 97,101.5 v97,102.15 | v94.47,122.67 94.47,128.77 v100.9,135.2 | v100.1,140.5 v100.1,138.28
!CLK_CAL  (via drill 0.2)
  Top 0.127: v76.45,138.5 76.6,138.35 76.6,127.8 75.78,126.98 58.62,126.98 56.1,124.45 56.1,102.1 54,100 44,100 43,99 43,98.3 34.3,89.6 34.3,75.1 43.15,66.25 43.15,21.5 42.45,20.8 42.45,19.2 42.6,19.05 45.5,19.05 45.9,19.45 45.9,20.01 46.9,21.01 47.91,21.01 49.35,22.45 49.35,22.55 U11.5 | v99.8,147.9 100.25,147.45 U31.81
  Bottom 0.127: v76.45,138.5 82.17,138.5 82.69,137.98 84.99,137.98 86.02,139.01 86.02,141.06 92.16,147.2 99.1,147.2 v99.8,147.9
!OUT_RANGE  (via drill 0.2)
  Top 0.127: U15.5 107.45,44.9 105.95,46.4 102.25,46.4 101.4,47.25 101.4,51.95 v102.15,52.7 | v101.5,56.17 101.5,57.3 94.54,64.26 92.93,64.26 92,65.18 92,67 86.5,72.5 86.5,83.45 83.7,86.25 83.7,95.55 v83.95,95.8 | v87.6,140.2 88.7,140.2 U31.10 | v84.85,131.15 84.22,130.52 84.22,128.77 84.46,128.53 v84.46,125.91
  Bottom 0.127: v84.85,131.15 85.34,131.64 85.44,131.64 87.6,133.8 v87.6,140.2 | v101.5,56.17 101.5,53.35 v102.15,52.7 | v83.95,95.8 83.95,110.87 83.71,111.1 83.71,113.92 82.69,114.94 82.69,121.34 84.48,123.14 84.48,125.89 v84.46,125.91
!PHY_RST  (via drill 0.2)
  Top 0.127: U32.15 140.75,132.42 139.33,131 125.51,131 v125.18,131.33 | U31.17 96.5,136.75 99.62,133.63 101.63,133.63 106.31,128.95 v108.6,128.95
  Bottom 0.127: v125.18,131.33 118.15,131.33 115.33,131.3 112.98,128.95 v108.6,128.95
!RF_OUT_EN  (via drill 0.2)
  Top 0.127: R82.1 69,28.6 74.35,33.95 | v74.35,34.85 74.35,33.95 | v74.65,36.3 74.65,41 74.25,41.4 74.25,42.1 U29.24 | v130.75,18.65 130.75,14.15 U18.9 | v127.45,26.15 127.45,32.95 125.85,34.55 125.15,34.55 U24.10 125.1,34.6 124.12,34.6 123.9,34.82 119.15,34.82 v117.85,33.52 | 74.35,33.95 74.9,33.95 75.45,33.4 89.15,33.4 96.15,40.4 v107.5,40.4
  Bottom 0.127: v74.35,34.85 74.65,35.15 v74.65,36.3 | v130.75,18.65 130.75,22.85 v127.45,26.15 | 107.6,40.4 v107.5,40.4 107.5,37.4 111.38,33.52 v117.85,33.52
!RIN_CTRL  (via drill 0.2)
  Top 0.127: v121.75,100.35 122.65,99.45 123.05,99.45 U4.24 | 113.65,107.65 v113.68,107.65 111.36,109.97 111.36,119.3 106.88,123.77 100.15,123.77 100.15,129.55 v100.2,129.6 | v101.7,135.2 101.7,137.58 v100.75,138.53 | v101.5,140.2 103,140.2 104.05,141.25 U31.68
  Bottom 0.127: v100.2,129.6 100.2,130.4 102.05,132.25 102.05,134.85 v101.7,135.2 | v100.75,138.53 100.75,139.45 v101.5,140.2 | v113.68,107.65 120.98,100.35 v121.75,100.35
!VCO_MON  (via drill 0.2)
  Top 0.127: R56.1 v83,21.33 | v83,21.33 R58.2 | U20.15 70.92,20.59 71.67,21.33 v73,21.33 | v83,21.33 | U29.26 75.21,38.12 v77,36.33
  Bottom 0.127: v73,21.33 v83,21.33 83,30.33 v77,36.33
!VCO_TUNE  (via drill 0.2)
  Top 0.127: v107.4,46.85 107.4,47.51 108.4,48.51 108.4,50.75 108.8,51.15 109.4,51.15 110.65,52.4 110.65,53.2 111.6,54.15 114.5,54.15 114.6,54.25 114.6,60.5 109.95,65.15 109.95,69.95 111,71 111,82 112,83 112,88.15 v111.95,88.2 | v97.45,101.7 96.8,101.7 93.05,105.45 93.05,121.99 92.93,122.11 92.11,122.11 VCO_TUNE.TP | v94.5,141.15 94.8,141.15 95.9,140.05 100.7,140.05 102.4,141.75 U31.69 | U10.5 97,17.1 97,18.25 98.89,20.14 99.25,20.14 99.58,20.48 99.58,24.83 100.45,25.7 v100.45,27.55
  Bottom 0.127: v100.45,27.55 101.8,28.9 101.8,41.25 v107.4,46.85 | v94.5,141.15 90.6,137.25 90.6,136.9 93.05,134.45 93.05,121.47 92.58,121 VCO_TUNE.TP | v97.45,101.7 106.15,93 109,93 111.95,90.05 v111.95,88.2
+3.3V  (via drill 0.71)
  Top 0.25: C144.1 R107.1 149,146.95 R111.1 R108.1 R109.1 | C126.1 87.2,138.25 U31.14 90.08,138.25 v90.33,138 | C129.1 99.25,148.8 U31.83 99.25,145.08 v99.33,145 | C128.1 94.25,148.8 U31.93 94.25,145.08 v94.33,145 | U31.74 107.33,144.25 | 107.33,144.25 108.3,144.25 C130.1 | C131.1 108.8,138.25 U31.62 103.25,138.25 v103,138 | C133.1 100.75,128.2 U31.46 100.75,132.42 v101,132.67 | C132.1 96.25,128.2 U31.37 96.25,132.58 v96.33,132.67 | U32.9 137.2,137.25 C137.2 | v107.33,145 107.33,144.25 | v103,133.33 103.08,133.25 U31.52 105.6,133.25 107.01,131.84 108.89,131.84 C134.1 | 125,98.05 C17.2 | U4.23 124.26,100.08 v124.67,99.67 | U7.23 102.59,88.92 103,89.33 103,90 | 103,90.95 C30.2 | C41.1 73.75,85.7 U9.18 73.75,89.81 v73.22,90.34 | U20.14 72,19.95 C72.1 | C108.2 66.71,40.04 U29.9 66.71,43.96 v66.67,44 | U29.1 61.22,42.11 v60.67,42.67 | U29.144 60.16,43.49 59.75,43.08 C116.2 | C117.2 58.07,46.96 U29.139 61.96,46.96 v62,47 | C102.2 73.71,40.04 U29.23 73.71,43.96 v73.67,44 | C103.2 77.71,39.96 U29.31 77.71,43.38 v78.33,44 | U29.37 81.86,43.39 C104.2 81.36,42.11 U29.36 80.21,43.79 80,44 v78.33,44 | v78.33,44 | C105.2 85.21,45.96 U29.40 80.04,45.96 v80,46 | C112.2 84.21,50.46 U29.49 80.13,50.46 v80,50.33 80.13,50.46 80.13,50.94 80.64,51.46 U29.51 | C114.2 85.21,59.46 U29.67 80.13,59.46 v80,59.33 | C115.2 81.86,63.11 U29.72 80.04,61.96 v80,62 80.21,62.21 U29.73 | C99.2 75.71,67.04 U29.82 75.71,62.04 v75.67,62 | C100.2 69.71,67.04 U29.94 69.71,62.04 v69.67,62 | C101.2 65.21,67.04 U29.103 65.21,62.21 v65,62 | C110.2 58.84,61.96 U29.109 61.96,61.96 v62,62 62.71,62.71 U29.108 61,63.91 | U29.117 59.09,57.96 58.8,58.25 C119.2 59.26,58.96 U29.115 62.04,58.96 v62.26,59.18
  Top 0.25: C118.2 58.08,52.46 U29.128 61.87,52.46 v62,52.33 | 104,60.95 L1.1 | U15.1 110.78,47.1 v110.98,47.3 | U12.27 103.19,58.35 102.91,58.62 102.91,61 v103.04,61.12 | R84.2A R84.3A R84.4A 50.22,51.78 v50.22,50.8 | 61,63.91 59.84,63.91 C106.2 | L6.2 61,63.91 | 103,90.95 103.05,90.95 | 103,90 103,90.95 | v104,90 103,90 | U30.3 60.07,133.01 61.46,134.4
  Top 0.5: SW1.D 6.5,29.5 5,28 5,24 SW1.C v38.33,22 | C9.+VE 38.05,124.95 C6.1 27.41,124.95 U1.3 SW2.SW2 | C96.2 146.95,26.25 U27.1 145.64,25.95 v145.54,26.05 | C97.2 146.95,33.25 U28.1 145.55,32.95 v145.54,32.97 | C42.1 95.03,13.07 U10.1 89.33,14.9 v88.89,15.33 | C98.2 R50.2 R52.2 R54.2 R56.2 C78.2 v85,27 | C75.2 61.95,18.9 R41.2 | U20.3 62.9,19.95 C75.2 | U20.6 62.9,18.05 C75.2 | C58.2 43.73,20.02 U16.5 45.38,22.07 U14.4 45.18,22.67 46.33,22.67 47.28,23.62 C50.2 47.38,23.67 47.38,24.38 v47.67,24.67 | 51.33,24.74 U11.1 51.46,24.62 C43.1 53.38,24.67 v54.58,24.67 | R82.2 R80.2 R81.2 R79.2 62.95,25 v61.67,25 | U26.1 146.65,46.7 C94.2 | C92.2 146.65,53.7 U25.1 145.75,51.95 v145.54,52.16 | U26.5 148.33,44 147.38,44.95 U26.1 | C145.1 160.25,140.16 P2.4 161.73,141.63 P2.5 | v38.33,22 | R85.2 R86.2 | R86.2 | R86.2 v55,148 | R104.1 R105.1 v127,144 | v127,144 | v137,133.67 137,134.95 C138.1 C137.2 | v149,148 149,146.95 | R112.1 v154,133 | v154,133 | L9.2 146.95,132.05 v147.33,131.67 | 96.05,128 C132.1 | 101.05,128 C133.1 | 125,98.05 125,99.33 v124.67,99.67 | 72,20.05 C72.1 72,19.95 v72,19 | v62,20 62,19.05 C75.2 | C116.2 60.5,42.5 v60.67,42.67 | C60.1 111.33,46.95 v110.98,47.3 | C44.1 102.92,61 v103.04,61.12 103.22,60.95 104,60.95 | U26.1 145.58,44.95 v145.54,45 | L8.1 87.41,127 v87.37,127.03 | P1.2 61.46,134.4 61.46,134.29 C123.1 | C30.2
  Bottom 0.5: SW4.SW2 14,69.46 14,95.54 | 14,95.54 14,122 12.46,123.54 SW2.SW2 | SW3.SW2 14,95.54
  other vias: 61.33,66.67
  pour Power: 48,68 68,68 68,92.26 73.77,92.26 73.77,68 144,68 148,64 148,22 144,22 144,52 137,59 113,59 113,46 109,46 109,59 87,59 87,17 90,17 90,14 38,14 38,29.67 48,29.67
  pour Power: 22,119 122,119 122,91 102,91 102,88 122,88 122,68 130,68 130,124 160,124 160,132 164,132 164,150 22,150
+3.3VF  (via drill 0.71)
  Top 0.25: C107.2 63,67.3 | U29.34 | 79.25,42.1 U29.34 | U29.143 63.11,44.96 63.21,45.06 | 59.75,41.05 C109.2 59.79,40.96 62.98,40.96 63.2,41.18 U29.2 63.21,45.06 | 64,46 63.92,46 63.21,45.29 63.21,45.06 | 79.87,40.7 79.87,40.96 79.71,41.12 U29.35 U29.34 | 79.87,40.7 79.87,39.88 C111.2 | 78,46 78,45.9 v78.34,45.57 | v80.38,40.7 79.87,40.7 | 78,60 78.42,60.42 79.87,60.42 80.92,61.46 U29.71 84.45,61.46 C113.2 | C107.2 63.21,67.04 U29.107 63.21,60.79 64,60 | L6.1 61.04,68.75 62.54,67.25 C107.2
  Top 1: 78,60 64,60 64,46 78,46
  Bottom 0.25: v78.34,45.57 80.38,43.52 v80.38,40.7
+5USB
  Top 0.178: R97.2 162.25,127 J8.1 161.5,120.75 D3.1
+5V  (via drill 0.71, 0.71 pad 0.2)
  Top 0.25: C39.1 75.25,98.8 U9.40 75.25,94.75 v75.33,94.67 | U9.47 71.75,98.8 C37.1 | U9.2 U9.3 | U9.2 68.42,94.25 67.9,94.77 C38.1 | C40.1 74.25,85.7 U9.19 74.25,90.1 v74.5,90.34 | U9.47 71.75,94.91 v71.72,94.88 | 69.89,93.95 69.89,94.01 U9.2 | U9.47 U9.46 U9.45 | 74.91,99.14 75.01,99.14 76.35,99.14 | 70.56,99.14 72,99.14 | U23.4 77.91,11.1 v79,10
  Top 0.5: U3.4 27.89,99.95 C10.1 41.95,99.95 C13.+VE v45,106 | C93.2 149.05,26.25 U27.6 150.43,25.95 v150.53,25.86 | C95.2 149.05,33.25 U28.6 150.45,32.95 v150.53,33.02 | C68.2 129,18.08 130.21,19.29 | 130.21,19.29 U18.8 | U23.4 75.79,11.1 C83.2 | C91.2 149.35,46.7 U26.6 150.42,44.95 v150.53,45.06 | C90.2 149.35,53.7 U25.6 150.25,51.95 v150.27,51.97 | U6.8 93,95.37 C27.1 91.85,96.05 v91.72,96.18 | U8.8 83.42,109.53 C32.1 83.02,109.93 v83.02,108.72 | 71.95,99 C37.1 72,99.14 | 68.1,94.77 C38.1 | v129.58,19.82 129.68,19.82 130.21,19.29 | U24.8 v130.86,36.21 130.06,37 C84.2 | v71.72,94.88 71.72,94.5 71.17,93.95 69.89,93.95 | L3.2 108.95,32.45 v111.75,35.25 | C39.1 75,99.13 75.01,99.14
  other vias: 117,97 116,98 117,100 116,96 117,94 135,97 136,98 136,96 135,94 135,95.5 70.73,98.99 76.11,99.25
  pour Power: 21,108 49,108 49,93 21,93
  pour Power: 49,100 76,100 76,112 94,112 105,101 118,101 118,93 78,93 78,88 74.51,88 74.51,93 49,93
  pour Power: 134.5,101 158,101 158,15 109.5,15 100.5,6 21,6 21,93 31,93 31,13 99,13 110,24 110.5,38 136,38 136,21 149,21 149,65 145,69 134.5,69
  pour Bottom: 115,101 115,93 137,93 137,101
+5VA
  Top 0.5: DIS1.VDD 17.41,144.95 C120.1 25.59,144.95 U2.3 27.41,145.95 C7.1 38.05,145.95 C11.+VE
+12V  (via drill 0.71)
  Top 0.25: U7.2 96.92,88.92 97,89 97,90.95 C28.1 | U5.8 C16.1
  Top 0.3: U4.2 130.97,100.08 C8.1
  Top 0.5: PWR1.+VOUT 39.13,85.95 C14.1 46.05,89 C18.+VE 47.2,89.15 v54.65,89.15 | U13.5 100.95,17.35 C49.1 101.1,19.2 101.1,24.11 103.79,26.8 108.15,26.8 110.05,28.7 114.4,28.7 115.46,27.65 v118.78,27.65 122.85,27.65 127.95,22.55 L2.2 | U17.7 123.03,54.63 122.88,54.78 | 122.88,54.78 122.88,57.93 C63.1 122.9,58.2 122.9,90.65 123,90.75 123,95.1 | R59.2 117.95,35.95 v117.95,36.25 | 97.28,96.28 96.95,95.95 96.95,91.05 C28.1 | 97.28,96.28 97.9,96.9 C16.1 98.25,97 100.3,94.95 103.45,94.95 103.9,95.4 109.75,95.4 110.05,95.1 123,95.1 | U4.2 128.8,100 128.16,100 127.74,99.58 127.74,96.77 126.08,95.1 123,95.1 | v63.42,96.2 65.3,96.2 84.9,115.8 90.7,115.8 91.8,114.7 91.8,101.75 97.28,96.28 | v122.8,53.95 122.8,54.55 122.88,54.78 | v122.62,49.15 v122.62,44.54
  Bottom 0.5: v122.8,53.95 122.8,49.33 v122.62,49.15 | 122.62,44.22 v122.62,44.54 122.62,40.92 120.06,38.36 120.06,36.35 | v54.65,89.15 56.37,89.15 v63.42,96.2 | v118.78,27.65 120.06,28.93 120.06,36.35 | v117.95,36.25 118.05,36.35 120.06,36.35
-12V  (via drill 0.71)
  Top 0.25: U4.21 122.04,101.38 122,101.33 | 122,101.33 | 122,101.33 121,100.33 121,100.05 C12.1 | C19.1 98,105.95 U5.3 98,101.33 97.68,101.02 97,100.33 U5.6 | U5.6
  Top 0.5: PWR1.-VOUT 39.03,75.95 C15.2 44.05,75.95 47,73 C20.-VE 47.15,71.8 47.15,41.25 62.6,25.8 72.6,25.8 73.6,24.8 86.2,24.8 86.8,24.2 C86.2 88.05,23 U22.2 90.56,23.1 U22.4 96.85,23.3 99.2,25.65 v99.2,27.3 | U17.4 119.47,50.42 C65.1 | 118.55,97.95 119.55,98.95 119.85,98.95 C12.1 | 118.55,97.95 117.35,97.95 113.8,101.5 104,101.5 103.45,100.95 97.75,100.95 97.68,101.02 | v100.6,28.7 102.9,31 102.9,35.5 103.45,36.05 104.85,36.05 109.8,41 109.8,41.95 111.25,43.4 114.57,43.4 115.2,44.03 115.2,45.57 119.04,49.41 C65.1 | v118.7,96 118.7,97.75 118.55,97.95 | v118.7,94.2 119.2,93.7 119.25,93.7 119.65,93.3 119.65,92.8 117.1,90.25 117.1,68.45 116.9,68.25 116.9,55.4 v116.95,55.35 | v116.95,52.65 119.15,50.45 C65.1
  Bottom 0.5: v99.2,27.3 v100.6,28.7 | v118.7,94.2 v118.7,96 | v116.95,52.65 v116.95,55.35
A0
  Top 0.127: U31.44 99.75,126.12 98.05,124.42 84.99,124.42 81.66,121.09 64.51,121.09 62,118.58 62,73.22 63.51,71.7 66.54,71.7 66.82,71.42 66.82,65.28 66.71,65.17 U29.100
A1
  Top 0.127: U31.43 99.25,126.13 97.79,124.67 84.74,124.67 81.41,121.34 64.26,121.34 61.74,118.83 61.74,72.96 63.26,71.45 66.28,71.45 66.56,71.17 66.56,65.54 66.21,65.19 U29.101
A4
  Top 0.127: U31.11 83.69,139.75 82.94,139.01 82.94,123.39 81.15,121.6 64,121.6 61.49,119.09 61.49,72.7 63,71.19 66.02,71.19 66.3,70.91 66.3,65.79 65.71,65.2 U29.102
A5
  Top 0.127: U31.2 83.58,144.25 81.15,141.82 81.15,125.18 79.36,123.39 62.21,123.39 59.7,120.88 59.7,72.75 55.3,68.35 55.3,60.42 55.55,60.16 58.62,60.16 59.32,59.46 U29.114
A6
  Top 0.127: U31.6 84.25,142.25 82.18,140.18 82.18,124.16 80.38,122.37 63.23,122.37 60.72,119.86 60.72,71.73 56.32,67.33 56.32,61.44 56.58,61.18 59.14,61.18 59.41,61.46 U29.110
ADC-BUSY
  Top 0.127: U9.29 79.76,91.25 80.13,90.88 80.13,76.8 81.41,75.52 81.41,68.1 78.21,64.9 U29.77
ADC-D0
  Top 0.127: U9.9 68.48,90.75 68.1,90.37 68.1,75.26 68.61,74.75 68.61,72.66 68.1,72.14 68.1,65.02 68.21,64.91 U29.97
ADC-D1
  Top 0.127: U9.10 68.49,90.25 68.35,90.11 68.35,75.52 68.86,75.01 68.86,72.4 68.35,71.89 68.35,65.28 68.71,64.92 U29.96
ADC-D2
  Top 0.127: U9.11 68.76,89.75 68.61,89.6 68.61,75.78 69.12,75.26 69.12,72.4 70.21,71.31 U29.93
ADC-D3
  Top 0.127: U9.12 69.03,89.25 68.86,89.09 68.86,76.03 69.38,75.52 69.38,72.66 70.71,71.32 U29.92
ADC-D4
  Top 0.127: U9.13 71.25,86.35 71.17,86.27 71.17,76.03 69.63,74.5 69.63,72.91 71.21,71.33 U29.91
ADC-D5
  Top 0.127: U9.14 71.75,86.34 71.42,86.02 71.42,77.82 74.24,75.01 74.24,72.19 71.71,69.66 U29.90
ADC-D6
  Top 0.127: U9.15 72.25,86.33 71.68,85.76 71.68,78.08 74.5,75.26 74.5,71.94 72.21,69.65 U29.89
ADC-D7
  Top 0.127: U9.16 72.75,86.32 71.94,85.5 71.94,78.34 74.75,75.52 74.75,71.68 72.71,69.64 U29.88
ADC-D8
  Top 0.127: U9.21 75.25,86.29 76.03,85.5 76.03,76.54 75.01,75.52 75.01,71.42 73.21,69.63 U29.87
ADC-D9
  Top 0.127: U9.22 75.75,86.3 76.29,85.76 76.29,76.29 75.26,75.26 75.26,71.17 73.71,69.61 U29.86
ADC-D10
  Top 0.127: U9.23 76.25,86.31 76.54,86.02 76.54,76.03 75.52,75.01 75.52,70.91 74.21,69.6 U29.85
ADC-D11
  Top 0.127: U9.24 76.75,86.58 76.8,86.53 76.8,75.78 75.78,74.75 75.78,70.66 74.71,69.59 U29.84
ADC-D12
  Top 0.127: U9.25 78.94,89.25 79.1,89.09 79.1,75.78 80.38,74.5 80.38,69.12 76.21,64.95 U29.81
ADC-D13
  Top 0.127: U9.26 79.21,89.75 79.36,89.6 79.36,76.03 80.64,74.75 80.64,68.86 76.71,64.93 U29.80
ADC-D14
  Top 0.127: U9.27 79.48,90.25 79.62,90.11 79.62,76.29 80.9,75.01 80.9,68.61 77.21,64.92 U29.79
ADC-D15
  Top 0.127: U9.28 79.75,90.75 79.87,90.62 79.87,76.54 81.15,75.26 81.15,68.35 77.71,64.91 U29.78
ADC_OB/!2C  (via drill 0.2)
  Top 0.127: U9.6 68.95,92.25 66.85,94.35 66.85,97.1 80.9,111.15 v84.4,111.15 | U31.96 v92.75,143.55 | v85.5,131.15 84.48,130.13 84.48,129.02 85.11,128.39 v85.11,125.91
  Bottom 0.127: v85.5,131.15 85.5,131.25 88.7,134.45 88.7,139.5 v92.75,143.55 | v84.4,111.15 84.4,113.74 82.94,115.2 82.94,121.09 85.11,123.26 v85.11,125.91
ADC_PD/!FD  (via drill 0.2)
  Top 0.127: U9.30 77.7,91.75 77.4,92.05 77.4,94.95 79.6,97.15 80.5,97.15 80.6,97.25 v80.6,101.39 | v86.25,123.95 86.25,117.55 85.59,116.89 81.09,116.89 v73.35,109.15 | v92.9,142.7 92.65,142.7 92.2,143.15 92.2,146.7 U31.97
  Bottom 0.127: v86.25,123.95 86.25,129.95 89,132.7 89,138.8 v92.9,142.7 | v80.6,101.39 73.35,108.64 v73.35,109.15
AGND  (via drill 0.2, 0.2 pad 0.2, 0.71)
  Top 1: 112.9,81.15 113,76.8
  other vias: 154,141 92.67,150.33 100.33,150.33 75,82 73,82 112,138 112.26,134.51 106.11,145.77 134.02,136.04 67.05,148.22 70.12,148.22 91.11,125.69 91.37,133.88 94.44,133.88 102.38,125.94 95.98,119.54 87.27,116.98 85.74,107 112.36,102.9 110.57,104.95 115.43,115.19 150.25,115.19 128.49,115.19 107.75,116.73 107.5,111.1 115.43,92.92 120.81,93.43 132.07,101.62 144.87,107.26 149.74,100.09 49.9,55.29 65.77,39.16 76.45,39.16 79.08,37.11 105.45,29.94 102.89,29.69 152.81,43 147.94,48.12 131.82,17.66 129.26,14.58 147.94,33.27 143.85,33.78 110.57,49.66 106.98,48.63 110.31,56.06 91.88,49.14 95.46,54.52 86.76,44.54 72.94,39.16 101.61,75.51 95.46,66.3 107.24,66.3 112.87,68.86 98.79,86.01 99.05,89.34 99.82,97.53 124.65,102.39 86.25,135.93 93.67,138.23 102.63,136.7 112.26,131.18 78.06,75.26 85.74,63.48 74.47,62.46 57.32,63.48 61.67,70.14 69.3,69.77 71.86,75.4 66.74,75.66 75.3,89.17 72.49,89.17 81.96,94.54 85.29,90.96 89.83,102.39 90.1,112.13 104.17,45.56 104.42,42.49 112.1,40.44 113.13,45.05 130.54,48.69 133.36,55.6 42.73,96.25 39.14,96.5 41.96,102.14 73.51,98.38 74.28,94.03 72.74,94.03 79.91,92.5 125.16,29.69 123.58,33.94 117.43,34.96 131.05,106.49 121.15,105.39 121.65,107.14 116.65,107.14 65,69.88 93.93,129.27 105.45,51.19 102.69,53.75 56.3,59.13 61.67,58.1 61.93,48.38 61.93,54.01 55.27,52.47 52.46,20.47 95.74,144.96 98.04,145.21 114.36,30.1 106.11,148.77 147.81,42 147.94,29.27 144.51,144.23 144,130.66 133.36,60.72 89.58,51.96 63,87 55,87 55,76 63,76 153.83,107.62 158,9 158,11 154,12 153,10 149,14 150,16 145,19 145,17 140,19 140,17 66.28,116.73 150.5,93.06 126.95,92.81 107.5,98.95 83.94,75.51 106.98,133.37 78.72,151.33 137.6,144.23 153.83,105.83 148.2,107.11 148.2,108.9 155.62,101.99 156.39,100.2 149.74,101.99 138.98,101.74 138.98,100.2 144.87,100.2 144.87,101.99 144.87,108.79 138.98,108.79 138.98,107.26 107.5,86.89 107.5,81 90.86,81 91.11,86.89 90.34,94.31 90.34,96.36 87.02,95.85 95.46,95.34 95.46,93.29 95.46,91.5 96.49,100.97 99.05,101.74 99.56,104.55 100.07,99.94 96.74,104.81 81.38,101.22 70.12,96.1 79.59,101.48 69.86,87.91 78.06,87.91 80.1,109.16 85.48,111.21 82.66,104.3 109.28,22.38 133.86,21.61 134.88,12.65 132.32,32.62 130.53,24.94 132.06,26.73 130.27,29.03 128.22,28.78 127.97,32.1 128.99,33.9 125.66,37.48 123.87,35.94 121.31,38.5 116.96,36.46 116.96,38.5 110.82,38.5 110.82,36.46 105,35.4 106.21,33.9 94.94,33.9 100.06,34.92 99.3,29.8 110.05,30.31 121.06,29.8 133.86,30.31 134.62,36.71 132.06,36.71 134.62,41.32 132.32,46.44 134.88,46.44 138.98,50.28 137.44,51.82 142.05,56.42 143.58,54.89 148.19,59.75 146.66,61.03 152.03,63.34 150.5,65.13 156.64,63.85 156.64,66.15 159.97,64.62 159.71,66.66 54.25,25.96 53.99,32.87 52.71,32.87 52.71,28.01 54.76,22.38 44.52,17.26 39.66,23.4 44.01,26.73 50.15,23.66 56.55,37.22 56.81,38.5 68.84,36.97 62.7,36.97 51.94,41.32 50.92,40.3 47.85,46.95 49.13,46.95 47.85,55.14 47.85,63.85 49.13,63.85 49.9,69.22 49.13,70.25 49.38,74.09 50.66,74.09 52.2,79.46 52.46,86.89 54.76,93.54 55.53,92.78 62.95,99.18 62.95,105.06 62.95,110.95 62.95,116.58 66.28,119.91 71.91,119.91 77.8,119.91 82.15,119.91 88.04,119.91 88.04,121.19 95.98,120.94 101.35,122.73 102.38,121.96 103.91,125.8 103.91,129.64 83.43,119.91 151,141 149,141
  pour Top (rank 5): 0,0 177,0 177,155.5 0,155.5
  pour Gnd (rank 5): 0,0 177,0 177,155.5 0,155.5
  pour Power (rank 5): 0,0 177,0 177,155.5 0,155.5
  pour Bottom (rank 5): 0,0 177,0 177,155.5 0,155.5
CONFIG_SEL  (via drill 0.2)
  Top 0.127: U29.126 59.18,53.46 v58.88,53.76 | R84.1B 51.87,54.27 v52.48,54.27
  Bottom 0.127: v58.88,53.76 52.99,53.76 v52.48,54.27
D0
  Top 0.127: U31.91 95.25,151.42 95,151.67 87.67,151.67 79.87,143.87 79.87,126.46 78.08,124.67 60.93,124.67 58.42,122.16 58.42,74.03 54.02,69.63 54.02,57.86 56.41,55.46 U29.122
D1
  Top 0.127: U31.94 93.75,147.58 92.67,148.67 85.33,148.67 80.13,143.46 80.13,126.21 78.34,124.42 61.18,124.42 58.67,121.9 58.67,73.78 54.27,69.38 54.27,58.11 56.42,55.96 U29.121
D2
  Top 0.127: U31.98 91.75,147.84 91.26,148.33 85.67,148.33 80.38,143.05 80.38,125.95 78.59,124.16 61.44,124.16 58.93,121.65 58.93,73.52 54.53,69.12 54.53,58.37 56.44,56.46 U29.120
D3
  Top 0.127: U31.99 91.25,147.67 90.92,148 86,148 80.64,142.64 80.64,125.7 78.85,123.9 61.7,123.9 59.18,121.39 59.18,73.26 54.78,68.86 54.78,58.62 56.45,56.96 U29.119
D4
  Top 0.127: U31.100 85.42,146.75 80.9,142.23 80.9,125.44 79.1,123.65 61.95,123.65 59.44,121.14 59.44,73.01 55.04,68.61 55.04,58.88 56.46,57.46 U29.118
D5
  Top 0.127: U31.3 83.75,143.75 81.41,141.41 81.41,124.93 79.62,123.14 62.46,123.14 59.95,120.62 59.95,72.5 55.55,68.1 55.55,60.67 55.81,60.42 58.88,60.42 59.34,59.96 U29.113
D6
  Top 0.127: U31.4 83.92,143.25 81.66,141 81.66,124.67 79.87,122.88 62.72,122.88 60.21,120.37 60.21,72.24 55.81,67.84 55.81,60.93 56.06,60.67 59.14,60.67 59.35,60.46 U29.112
D7
  Top 0.127: U31.5 84.08,142.75 81.92,140.59 81.92,124.42 80.13,122.62 62.98,122.62 60.46,120.11 60.46,71.98 56.06,67.58 56.06,61.18 56.32,60.93 59.39,60.93 59.42,60.96 U29.111
D8
  Top 0.127: U31.88 96.75,150.58 95.33,152 87.33,152 79.62,144.28 79.62,126.72 77.82,124.93 60.67,124.93 58.16,122.42 58.16,74.29 53.76,69.89 53.76,57.6 56.4,54.96 U29.123
D9
  Top 0.127: U31.87 97.25,150.75 95.67,152.33 87,152.33 79.36,144.69 79.36,126.98 77.57,125.18 60.42,125.18 57.9,122.67 57.9,74.54 53.5,70.14 53.5,57.34 56.39,54.46 U29.124
D10
  Top 0.127: U31.86 97.75,147.92 97.67,148 97.67,151 96,152.67 86.67,152.67 79.1,145.1 79.1,127.23 77.31,125.44 60.16,125.44 57.65,122.93 57.65,74.8 53.25,70.4 53.25,57.09 56.32,54.02 57.86,54.02 58.91,52.96 U29.127
D11
  Top 0.127: U31.85 98.25,148.08 98,148.33 98,151.33 96.33,153 86.33,153 78.85,145.51 78.85,127.49 77.06,125.7 59.9,125.7 57.39,123.18 57.39,75.06 52.99,70.66 52.99,56.83 54.53,55.3 54.53,51.97 55.3,51.2 58.88,51.2 59.14,51.46 U29.130
D12
  Top 0.127: U29.132 59.36,50.46 59.14,50.69 54.78,50.69 54.02,51.46 54.02,54.78 52.48,56.32 52.48,71.17 56.88,75.57 56.88,123.7 59.39,126.21 76.54,126.21 78.34,128 78.34,146.34 85.67,153.67 99.33,153.67 101.38,151.62 101.38,147.71 101.25,147.59 U31.79
D13
  Top 0.127: U31.80 100.75,147.6 101.12,147.97 101.12,151.3 99.08,153.33 86,153.33 78.59,145.93 78.59,127.74 76.8,125.95 59.65,125.95 57.14,123.44 57.14,75.31 52.74,70.91 52.74,56.58 54.27,55.04 54.27,51.71 55.04,50.94 59.14,50.94 59.15,50.96 U29.131
D14
  Top 0.127: U31.77 102.25,147.57 101.89,147.93 101.89,152.44 100,154.33 85,154.33 77.82,147.16 77.82,128.51 76.03,126.72 58.88,126.72 56.37,124.21 56.37,76.08 51.97,71.68 51.97,55.81 53.5,54.27 53.5,50.94 54.27,50.18 57.6,50.18 58.82,48.96 U29.135
D15
  Top 0.127: U29.134 58.83,49.46 57.86,50.43 54.53,50.43 53.76,51.2 53.76,54.53 52.22,56.06 52.22,71.42 56.62,75.82 56.62,123.95 59.14,126.46 76.29,126.46 78.08,128.26 78.08,146.75 85.33,154 99.67,154 101.63,152.03 101.63,147.71 101.75,147.59 U31.78
DAC0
